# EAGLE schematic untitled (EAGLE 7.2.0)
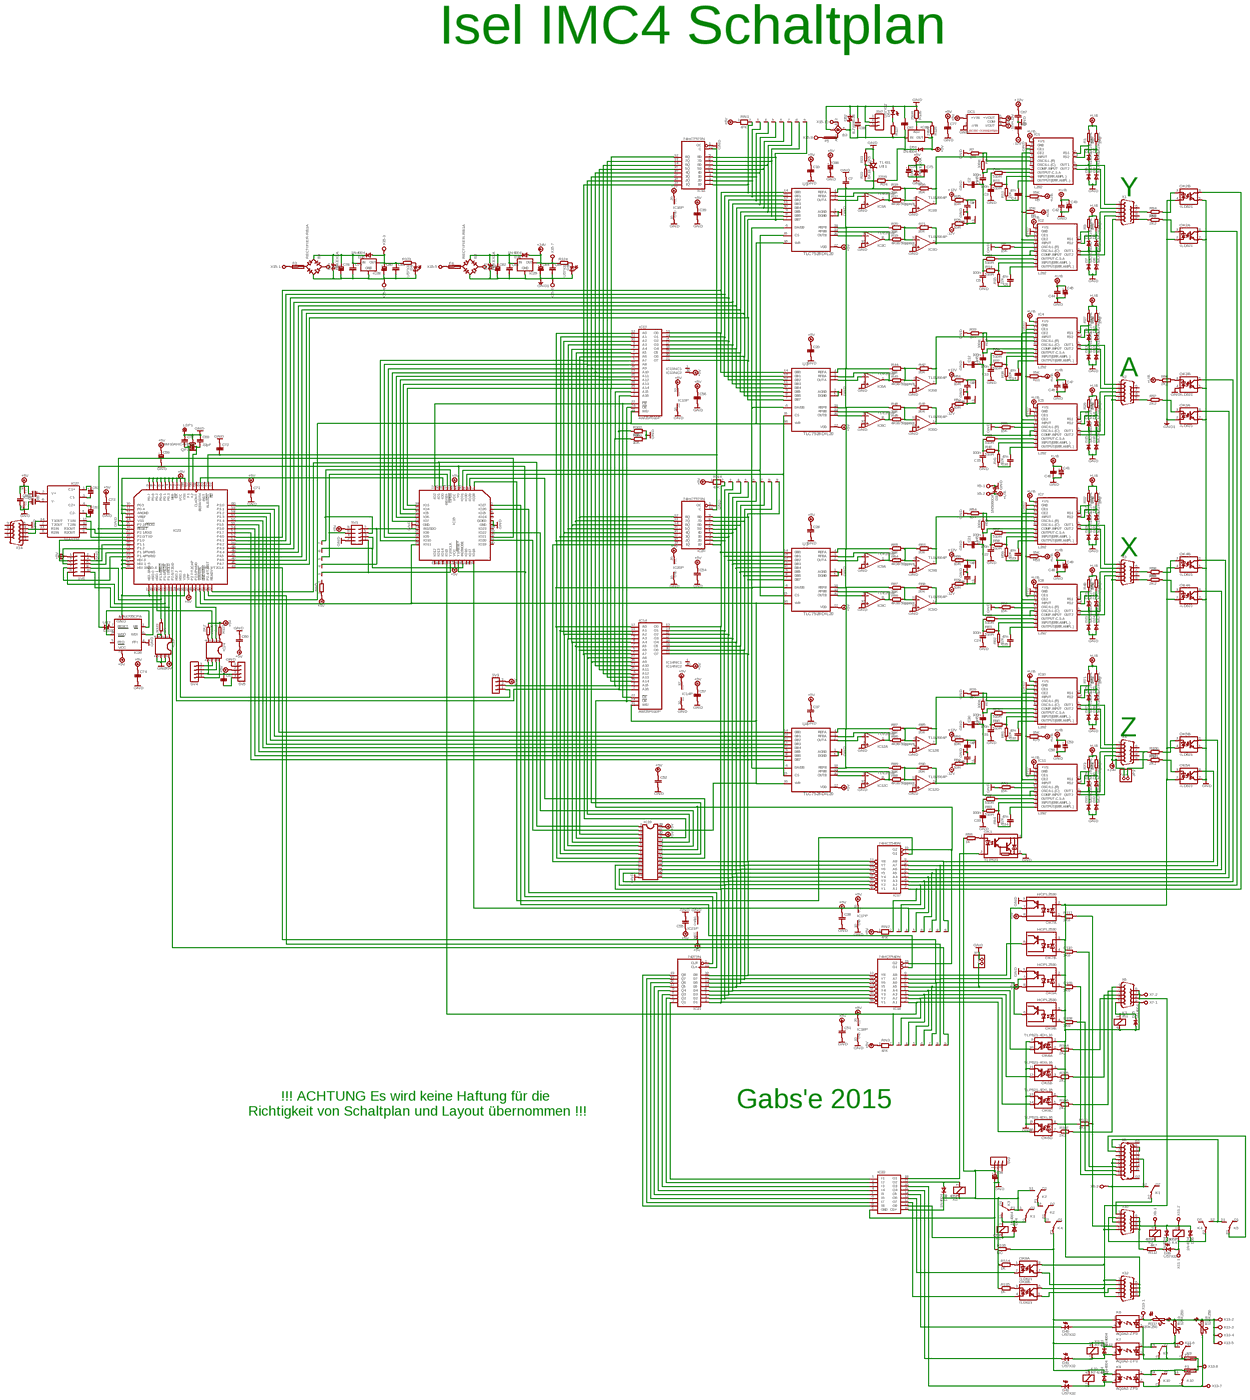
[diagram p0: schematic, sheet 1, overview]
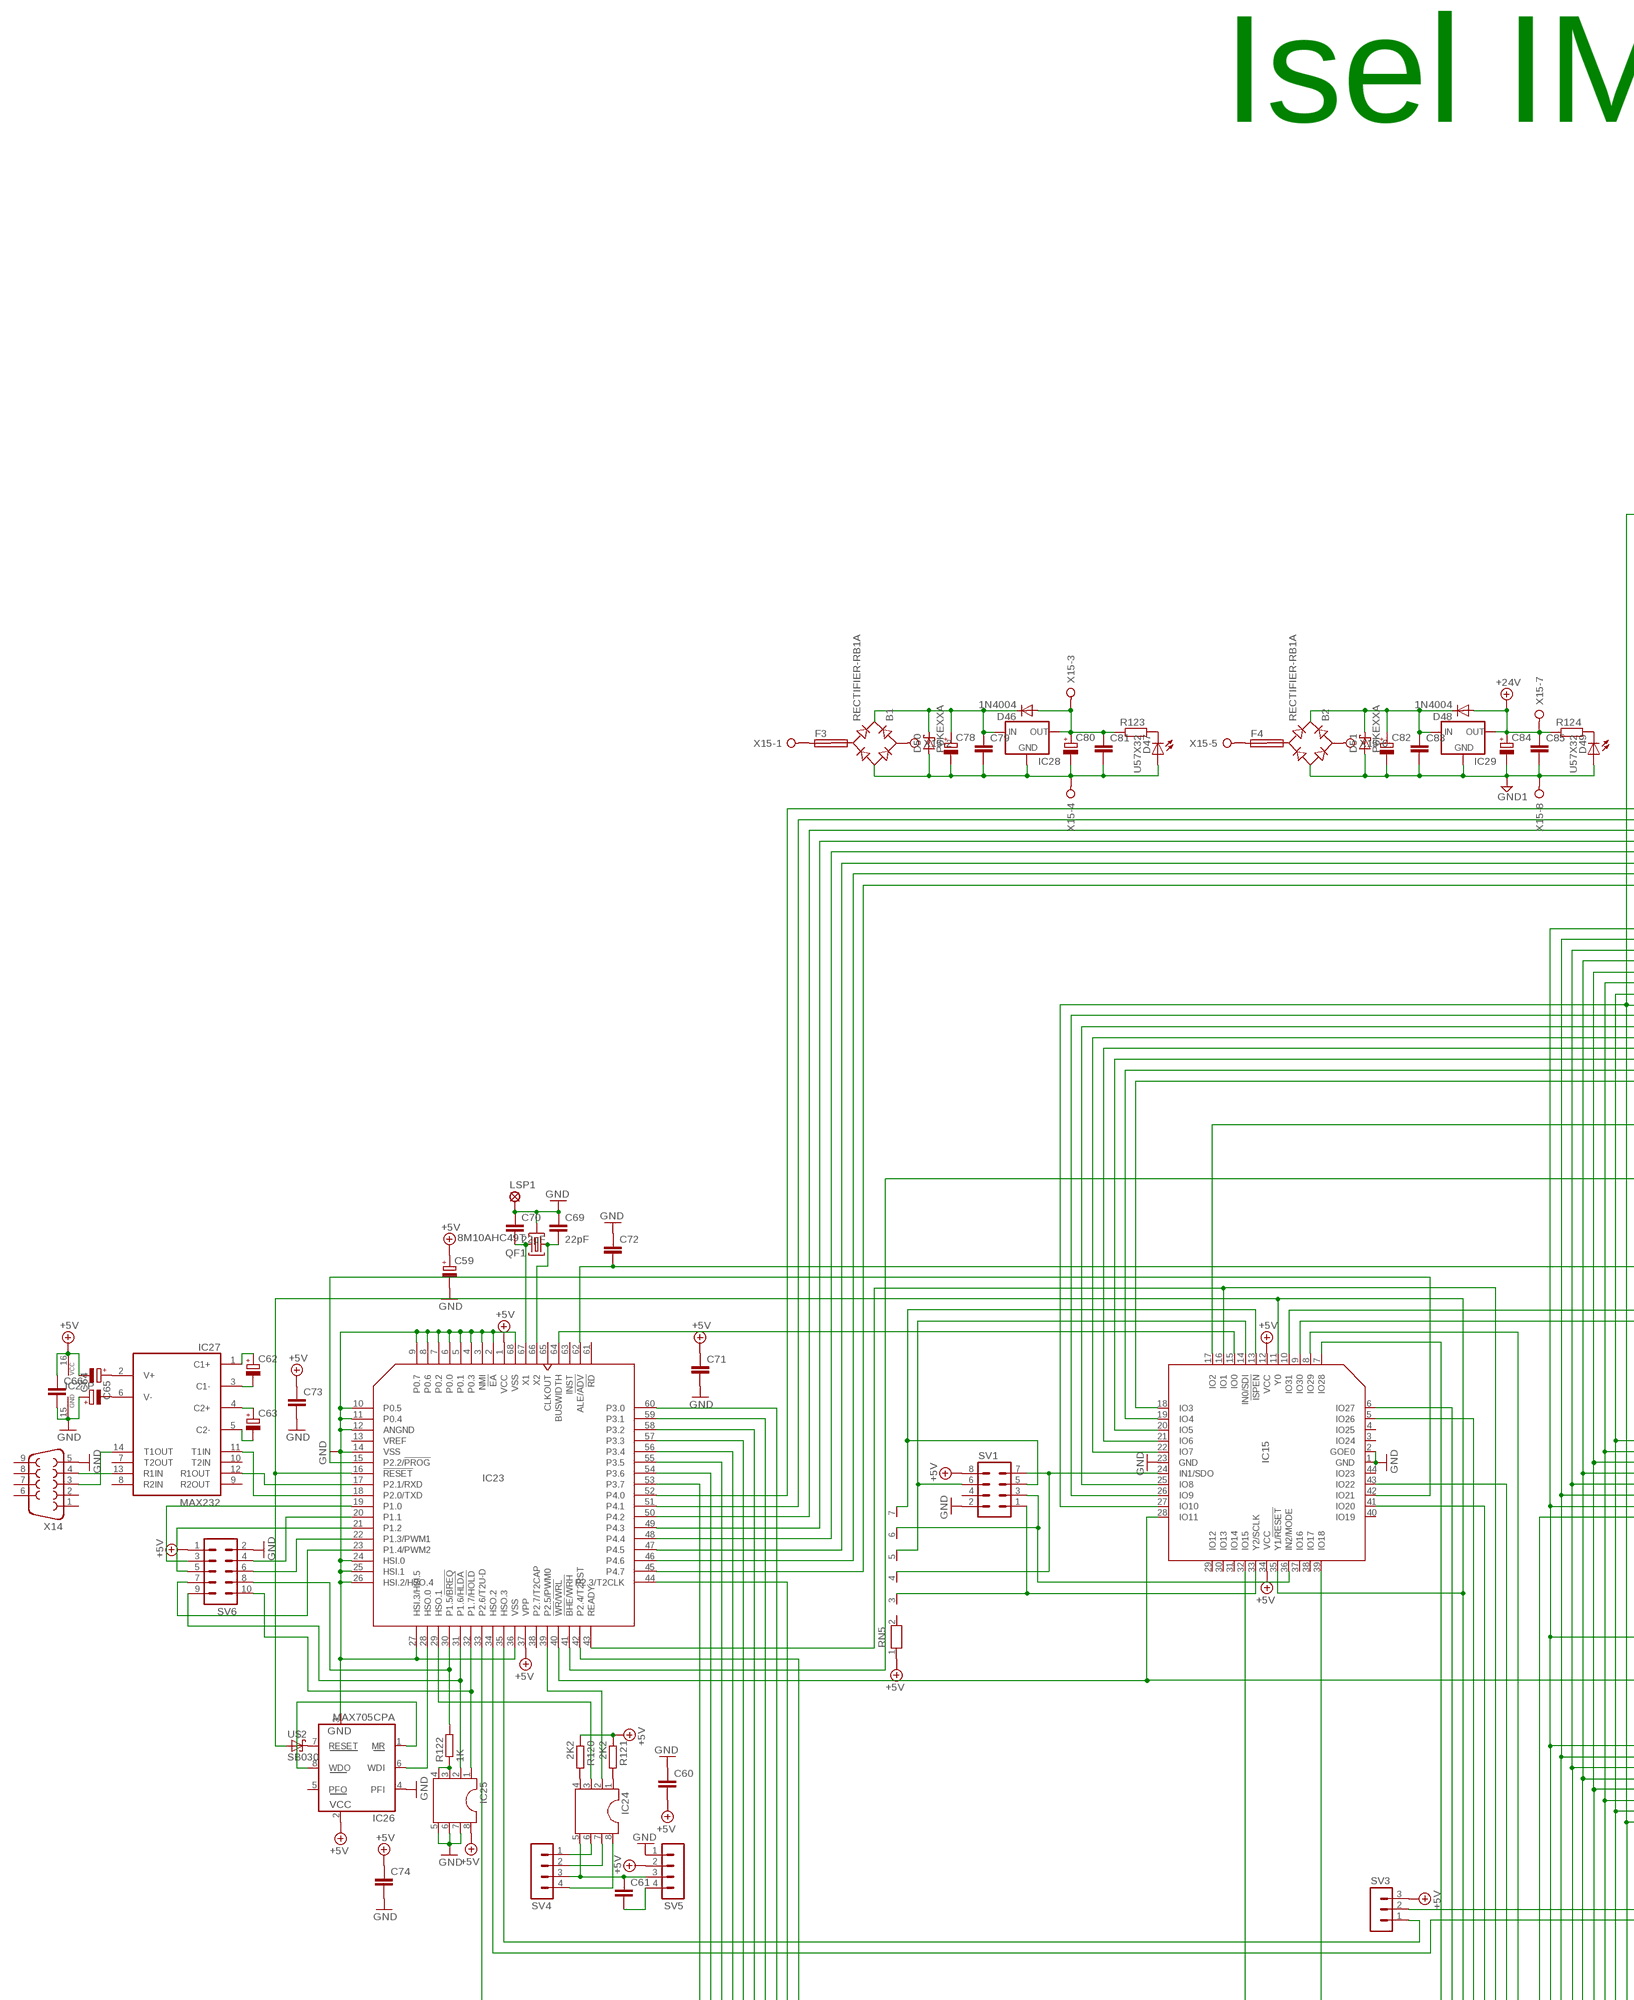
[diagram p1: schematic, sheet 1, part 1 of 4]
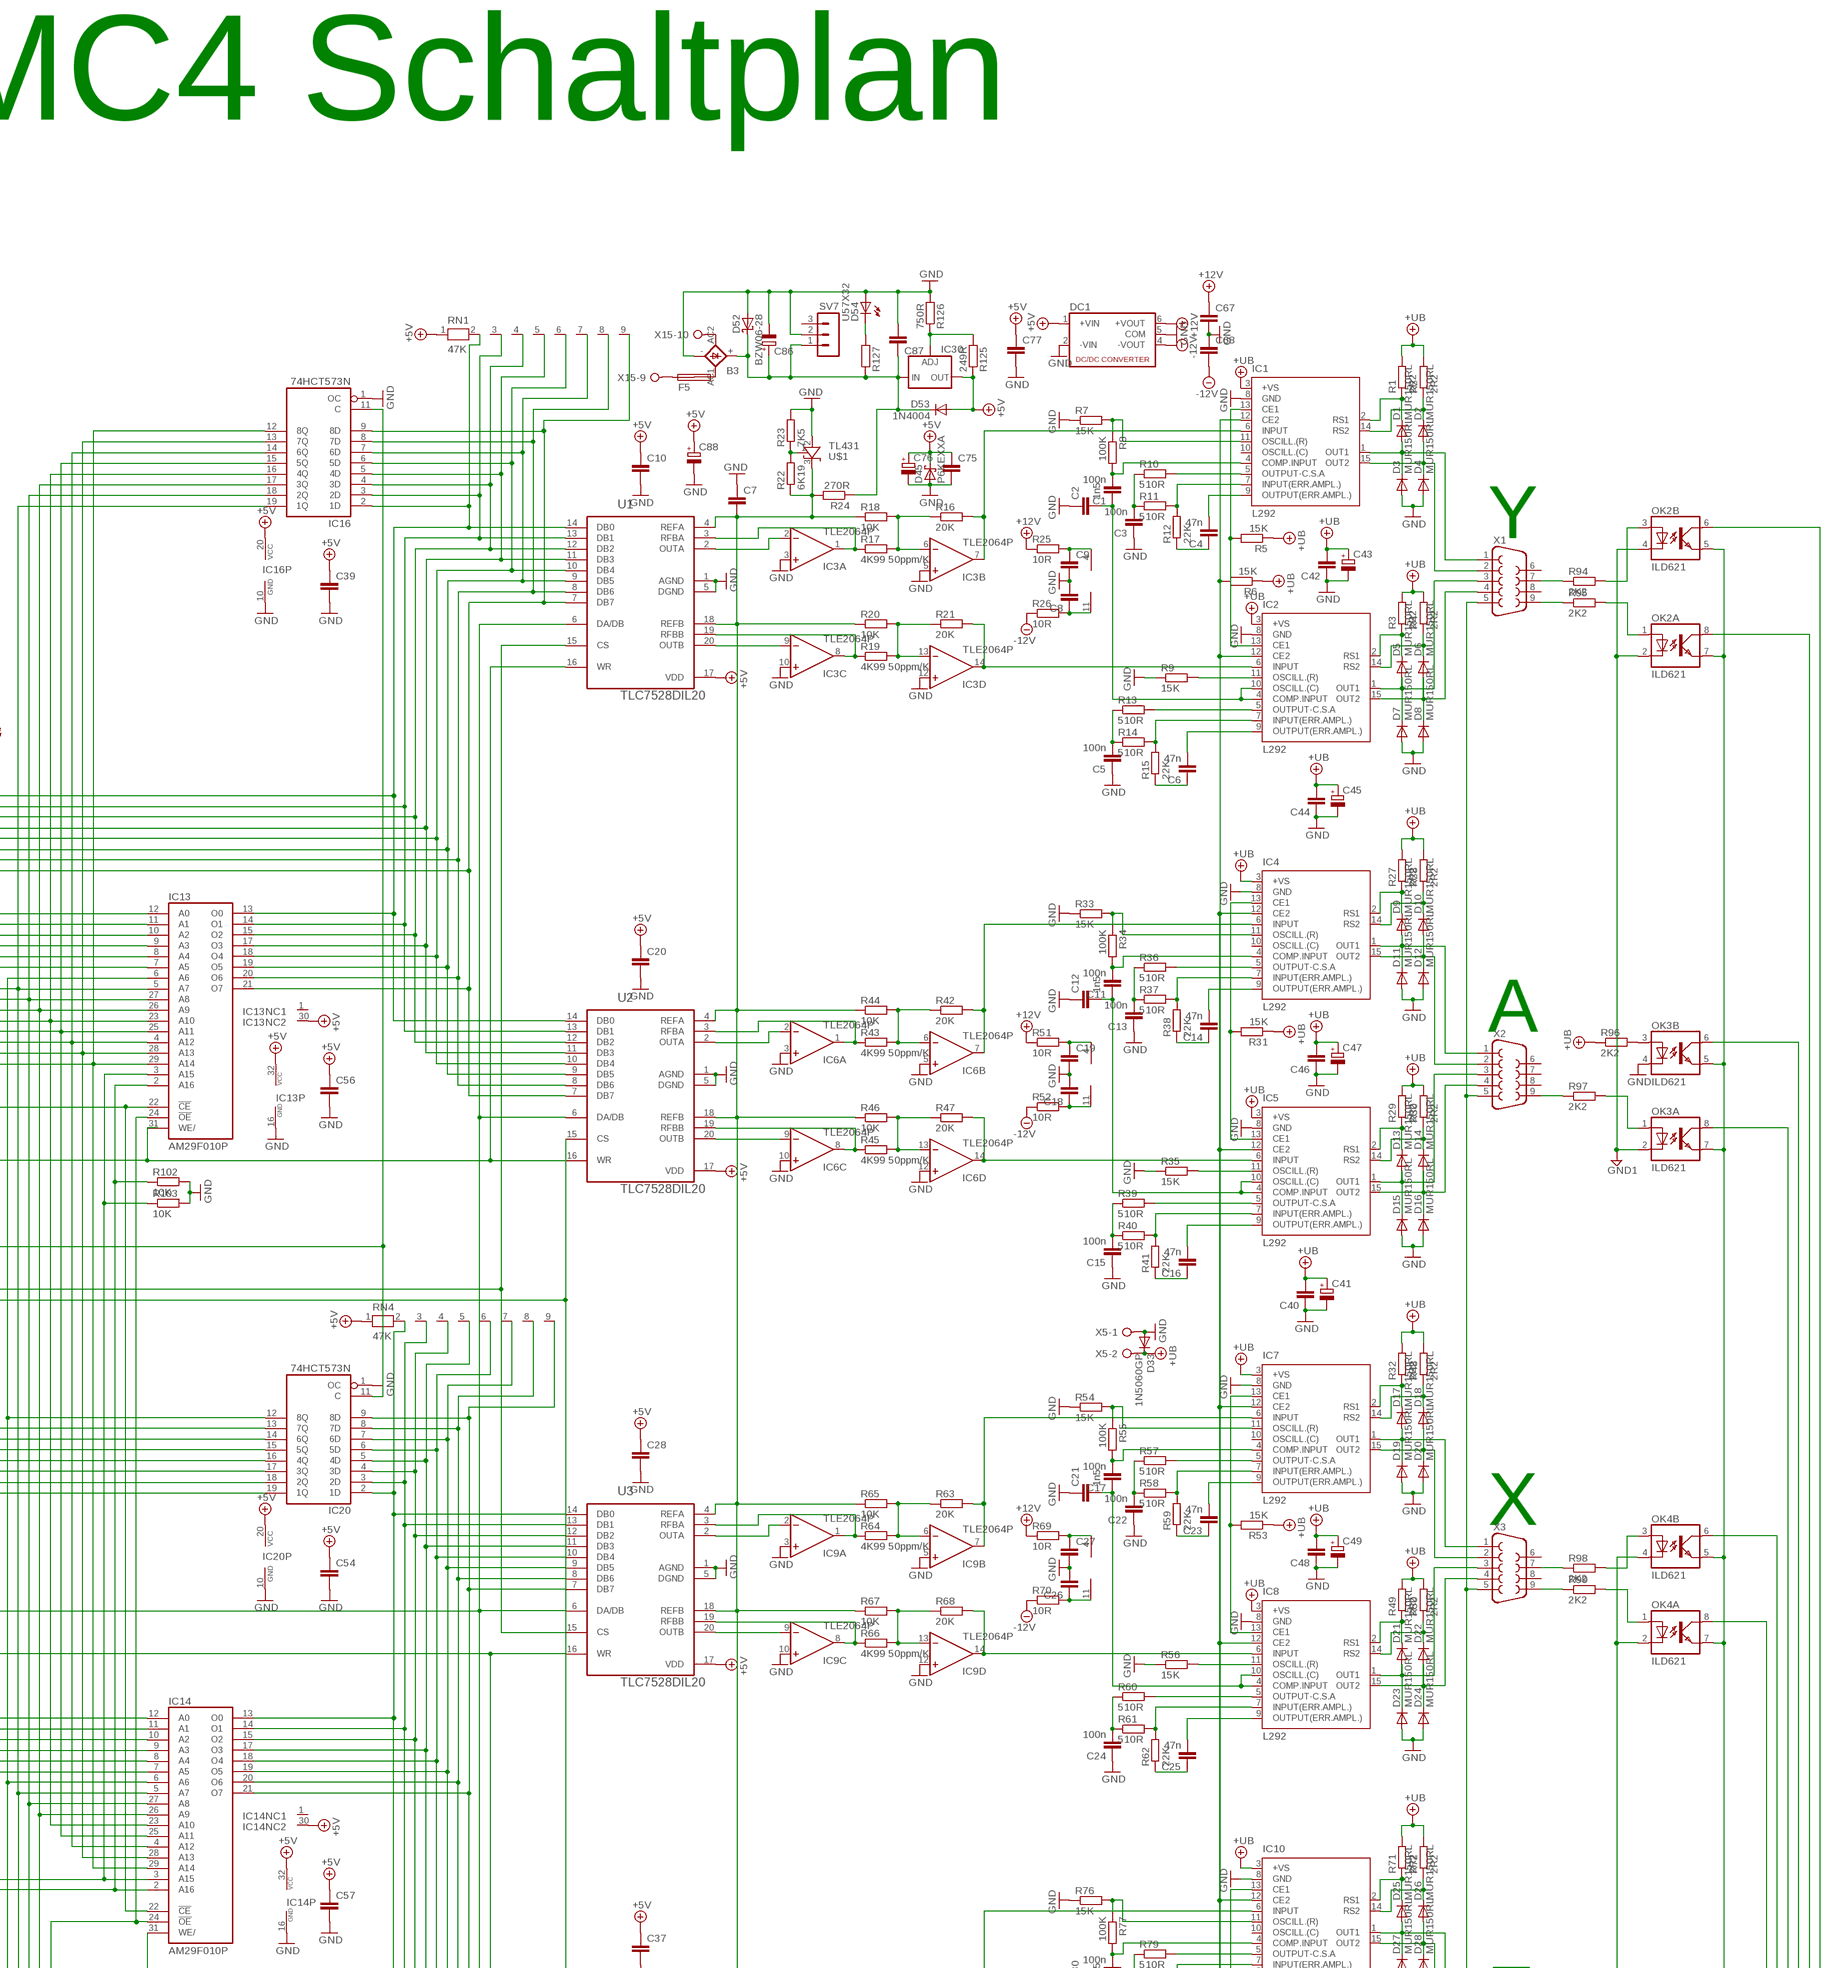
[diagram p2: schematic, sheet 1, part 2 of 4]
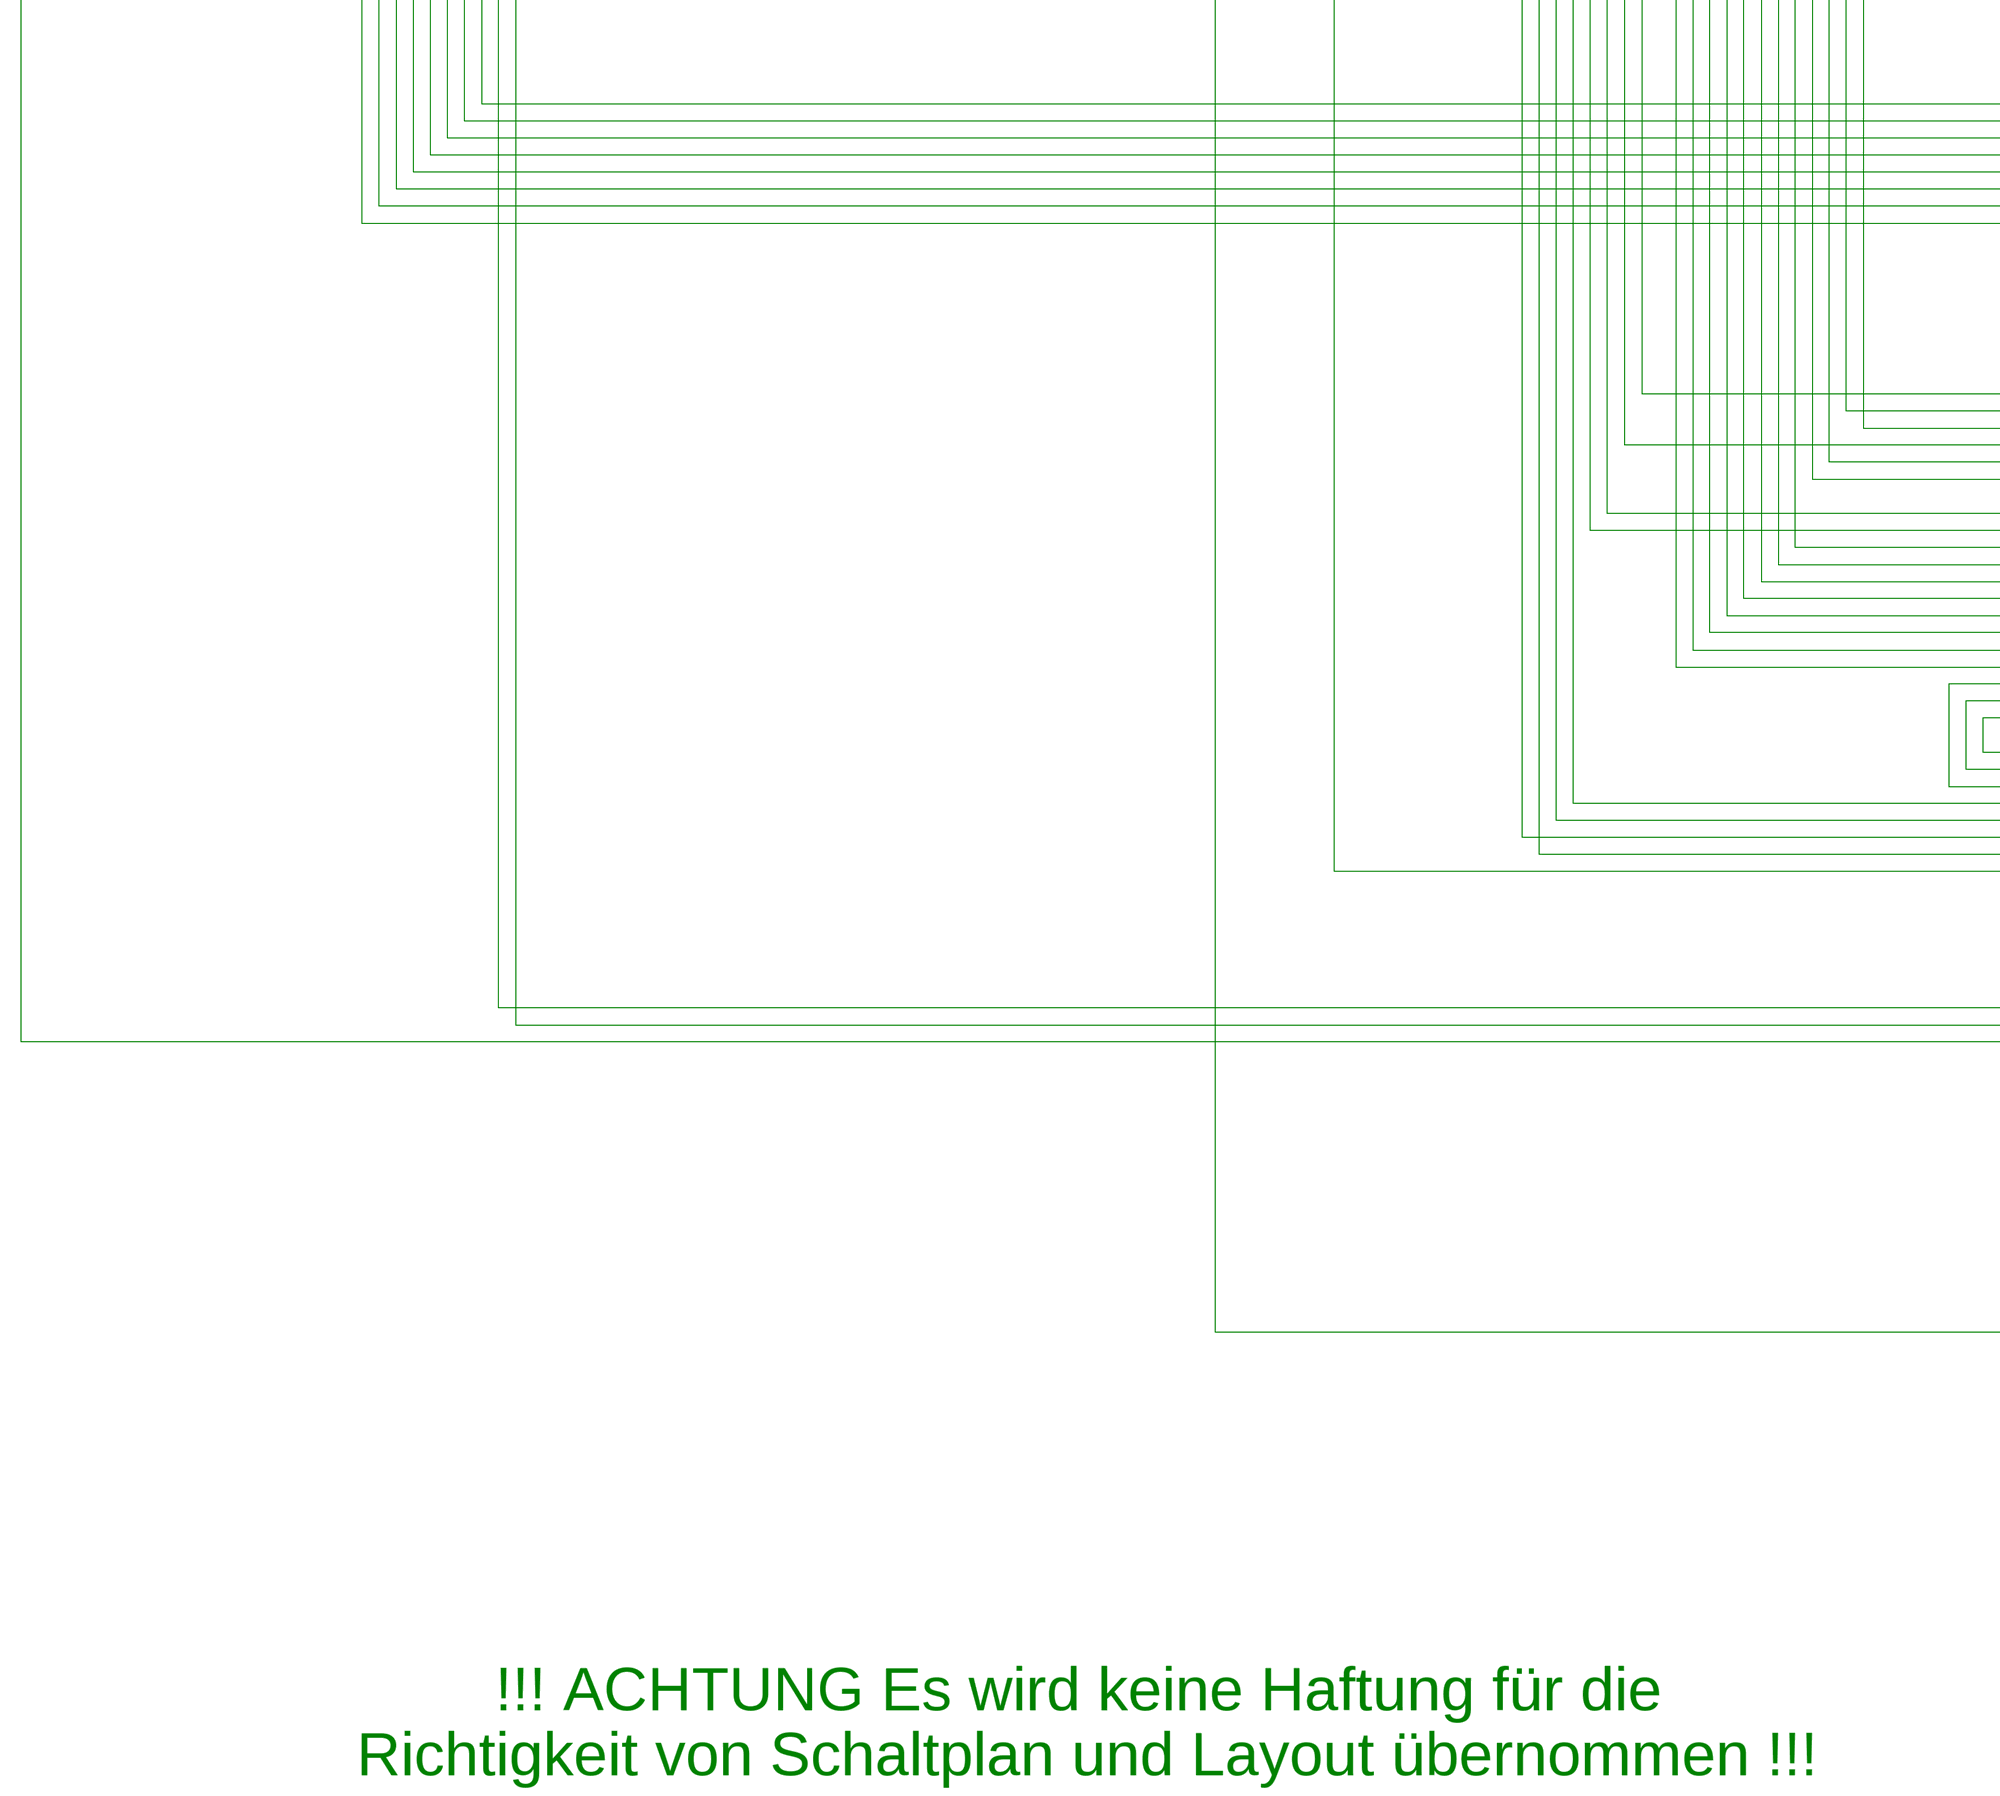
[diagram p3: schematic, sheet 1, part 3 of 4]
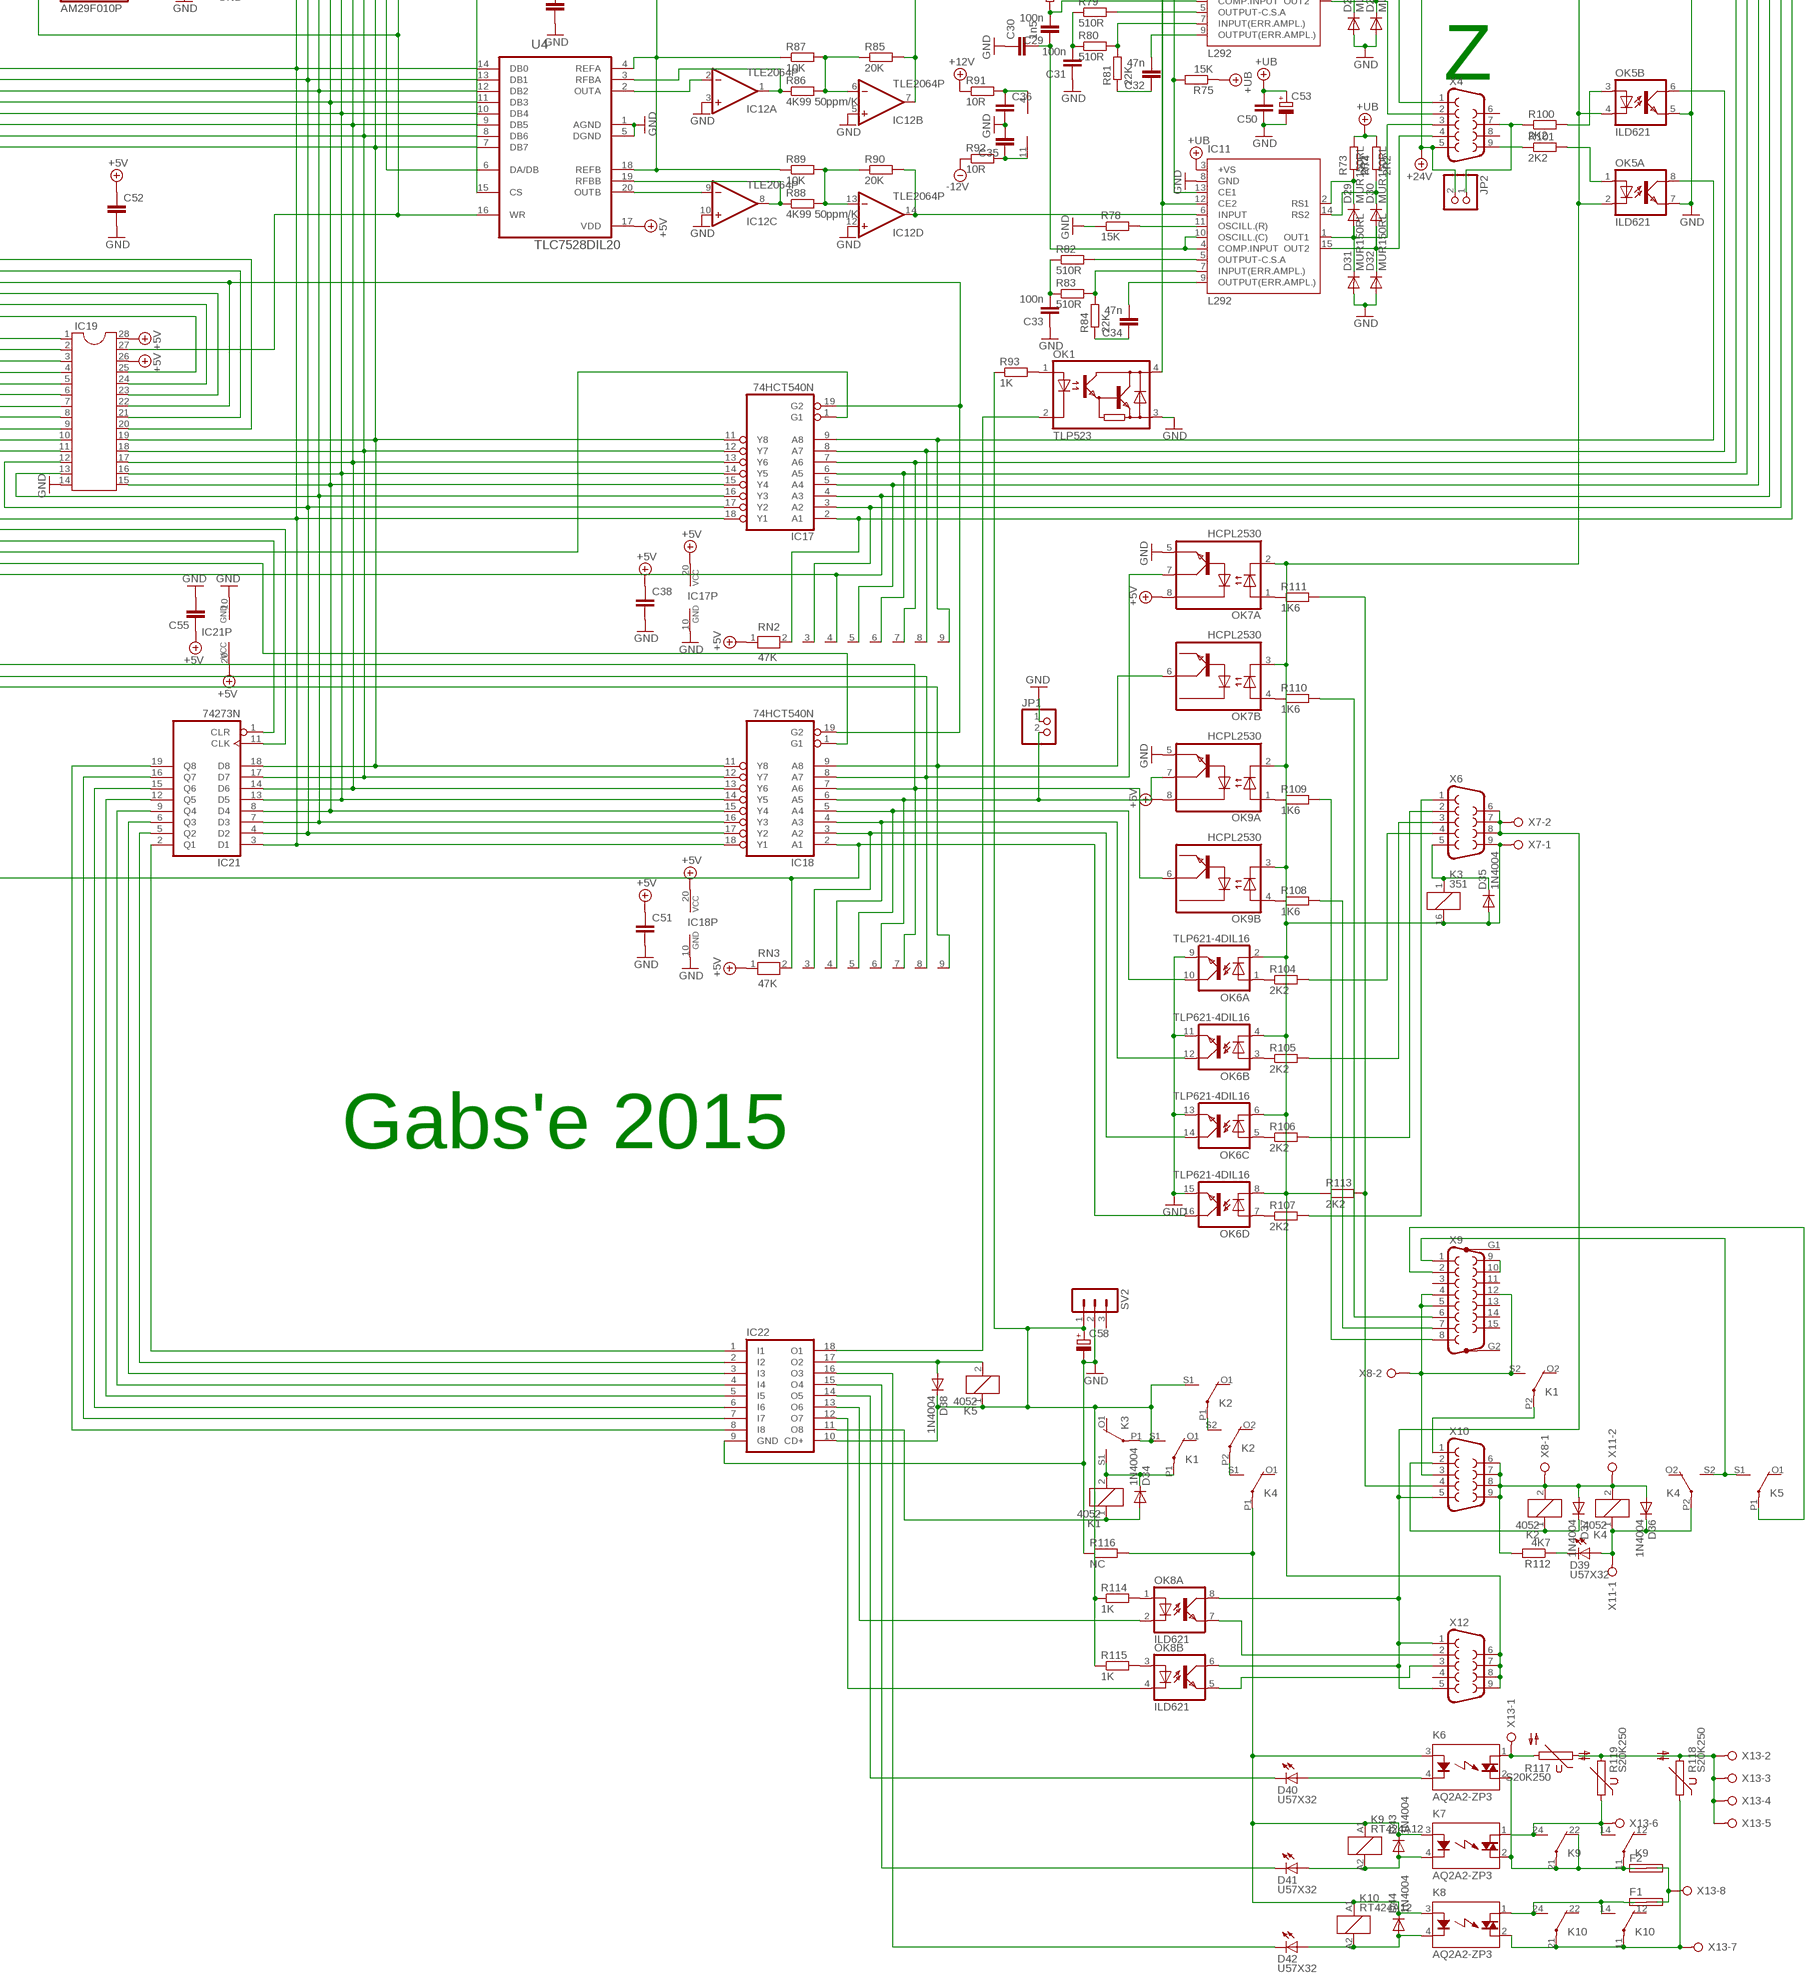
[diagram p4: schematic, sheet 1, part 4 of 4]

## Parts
B1  RECTIFIER-RB1A  [RB1A]
B2  RECTIFIER-RB1A  [RB1A]
B3  2KBB-R  [2KBB-R]
C1  100n  C-EU050-025X075  [C050-025X075]
C2  1n5  C-EU050-025X075  [C050-025X075]
C3  100n  C-EU050-025X075  [C050-025X075]
C4  47n  C-EU050-025X075  [C050-025X075]
C5  100n  C-EU050-025X075  [C050-025X075]
C6  47n  C-EU050-025X075  [C050-025X075]
C7  C-EU025-024X044  [C025-024X044]
C8  C-EU025-024X044  [C025-024X044]
C9  C-EU025-024X044  [C025-024X044]
C10  C-EU025-024X044  [C025-024X044]
C11  100n  C-EU050-025X075  [C050-025X075]
C12  1n5  C-EU050-025X075  [C050-025X075]
C13  100n  C-EU050-025X075  [C050-025X075]
C14  47n  C-EU050-025X075  [C050-025X075]
C15  100n  C-EU050-025X075  [C050-025X075]
C16  47n  C-EU050-025X075  [C050-025X075]
C17  100n  C-EU050-025X075  [C050-025X075]
C18  C-EU025-024X044  [C025-024X044]
C19  C-EU025-024X044  [C025-024X044]
C20  C-EU025-024X044  [C025-024X044]
C21  1n5  C-EU050-025X075  [C050-025X075]
C22  100n  C-EU050-025X075  [C050-025X075]
C23  47n  C-EU050-025X075  [C050-025X075]
C24  100n  C-EU050-025X075  [C050-025X075]
C25  47n  C-EU050-025X075  [C050-025X075]
C26  C-EU025-024X044  [C025-024X044]
C27  C-EU025-024X044  [C025-024X044]
C28  C-EU025-024X044  [C025-024X044]
C29  100n  C-EU050-025X075  [C050-025X075]
C30  1n5  C-EU050-025X075  [C050-025X075]
C31  100n  C-EU050-025X075  [C050-025X075]
C32  47n  C-EU050-025X075  [C050-025X075]
C33  100n  C-EU050-025X075  [C050-025X075]
C34  47n  C-EU050-025X075  [C050-025X075]
C35  C-EU025-024X044  [C025-024X044]
C36  C-EU025-024X044  [C025-024X044]
C37  C-EU025-024X044  [C025-024X044]
C38  C-EU025-024X044  [C025-024X044]
C39  C-EU025-024X044  [C025-024X044]
C40  C-EU025-024X044  [C025-024X044]
C41  CPOL-EUE2.5-6  [E2,5-6]
C42  C-EU050-025X075  [C050-025X075]
C43  CPOL-EUE2,5-6E  [E2,5-6E]
C44  C-EU050-025X075  [C050-025X075]
C45  CPOL-EUE2.5-6  [E2,5-6]
C46  C-EU050-025X075  [C050-025X075]
C47  CPOL-EUE2.5-6  [E2,5-6]
C48  C-EU050-025X075  [C050-025X075]
C49  CPOL-EUE2.5-6  [E2,5-6]
C50  C-EU050-025X075  [C050-025X075]
C51  C-EU025-024X044  [C025-024X044]
C52  C-EU025-024X044  [C025-024X044]
C53  CPOL-EUE2.5-6  [E2,5-6]
C54  C-EU025-024X044  [C025-024X044]
C55  C-EU025-024X044  [C025-024X044]
C56  C-EU025-024X044  [C025-024X044]
C57  C-EU025-024X044  [C025-024X044]
C58  CPOL-EUE1.8-4  [E1,8-4]
C59  CPOL-EUE2.5-6  [E2,5-6]
C60  C-EU025-024X044  [C025-024X044]
C61  C-EU025-024X044  [C025-024X044]
C62  CPOL-EUE2.5-6  [E2,5-6]
C63  CPOL-EUE2.5-6  [E2,5-6]
C64  CPOL-EUE2,5-6E  [E2,5-6E]
C65  CPOL-EUE2.5-6  [E2,5-6]
C66  C-EU025-024X044  [C025-024X044]
C67  C-EU025-024X044  [C025-024X044]
C68  C-EU025-024X044  [C025-024X044]
C69  22pF  C-EU025-024X044  [C025-024X044]
C70  22pF  C-EU025-024X044  [C025-024X044]
C71  C-EU025-024X044  [C025-024X044]
C72  C-EU025-024X044  [C025-024X044]
C73  C-EU025-024X044  [C025-024X044]
C74  C-EU025-024X044  [C025-024X044]
C75  C-EU025-024X044  [C025-024X044]
C76  CPOL-EUE2.5-6  [E2,5-6]
C77  C-EU025-024X044  [C025-024X044]
C78  CPOL-EUE7.5-16  [E7,5-16]
C79  C-EU025-024X044  [C025-024X044]
C80  CPOL-EUE2-5  [E2-5]
C81  C-EU025-024X044  [C025-024X044]
C82  CPOL-EUE7.5-16  [E7,5-16]
C83  C-EU025-024X044  [C025-024X044]
C84  CPOL-EUE2-5  [E2-5]
C85  C-EU025-024X044  [C025-024X044]
C86  CPOL-EUE7.5-16  [E7,5-16]
C87  C-EU025-024X044  [C025-024X044]
C88  CPOL-EUE2.5-6  [E2,5-6]
D1  MUR150RL  [DO41-10]
D2  MUR150RL  [DO41-10]
D3  MUR150RL  [DO41-10]
D4  MUR150RL  [DO41-10]
D5  MUR150RL  [DO41-10]
D6  MUR150RL  [DO41-10]
D7  MUR150RL  [DO41-10]
D8  MUR150RL  [DO41-10]
D9  MUR150RL  [DO41-10]
D10  MUR150RL  [DO41-10]
D11  MUR150RL  [DO41-10]
D12  MUR150RL  [DO41-10]
D13  MUR150RL  [DO41-10]
D14  MUR150RL  [DO41-10]
D15  MUR150RL  [DO41-10]
D16  MUR150RL  [DO41-10]
D17  MUR150RL  [DO41-10]
D18  MUR150RL  [DO41-10]
D19  MUR150RL  [DO41-10]
D20  MUR150RL  [DO41-10]
D21  MUR150RL  [DO41-10]
D22  MUR150RL  [DO41-10]
D23  MUR150RL  [DO41-10]
D24  MUR150RL  [DO41-10]
D25  MUR150RL  [DO41-10]
D26  MUR150RL  [DO41-10]
D27  MUR150RL  [DO41-10]
D28  MUR150RL  [DO41-10]
D29  MUR150RL  [DO41-10]
D30  MUR150RL  [DO41-10]
D31  MUR150RL  [DO41-10]
D32  MUR150RL  [DO41-10]
D33  1N5060GP  [DO15-12]
D34  1N4004  [DO41-10]
D35  1N4004  [DO41-10]
D36  1N4004  [DO41-10]
D37  1N4004  [DO41-10]
D38  1N4004  [DO41-10]
D39  U57X32  [U57X32]
D40  U57X32  [U57X32]
D41  U57X32  [U57X32]
D42  U57X32  [U57X32]
D43  1N4004  [DO41-10]
D44  1N4004  [DO41-10]
D45  P6KEXXA  [C1702-15]
D46  1N4004  [DO41-10]
D47  U57X32  [U57X32]
D48  1N4004  [DO41-10]
D49  U57X32  [U57X32]
D50  P6KEXXA  [C1702-15]
D51  P6KEXXA  [C1702-15]
D52  BZW06-28  [P1-12E]
D53  1N4004  [DO41-10]
D54  U57X32  [U57X32]
DC1  NMA  [NMA]
F1  SHK20L  [SHK20L]
F2  SHK20L  [SHK20L]
F3  SHK20L  [SHK20L]
F4  SHK20L  [SHK20L]
F5  SHK20L  [SHK20L]
IC1  L292  [MULTIWATT-15]
IC2  L292  [MULTIWATT-15]
IC3  TLE2064P  [DIL14]
IC4  L292  [MULTIWATT-15]
IC5  L292  [MULTIWATT-15]
IC6  TLE2064P  [DIL14]
IC7  L292  [MULTIWATT-15]
IC8  L292  [MULTIWATT-15]
IC9  TLE2064P  [DIL14]
IC10  L292  [MULTIWATT-15]
IC11  L292  [MULTIWATT-15]
IC12  TLE2064P  [DIL14]
IC13  AM29F010P  [DIL32-3]
IC14  AM29F010P  [DIL32-3]
IC15  LSI2032PLCC  [S44]
IC16  74HCT573N  [DIL20]
IC17  74HCT540N  [DIL20]
IC18  74HCT540N  [DIL20]
IC19  DIL28  [DIL28-6]
IC20  74HCT573N  [DIL20]
IC21  74273N  [DIL20]
IC22  ULN2803A  [DIL18]
IC23  N80C196KC  [S68]
IC24  DIL8  [DIL08]
IC25  DIL8  [DIL08]
IC26  MAX705CPA  [DIL08]
IC27  MAX232  [DIL16]
IC28  78XXS  [78XXS]
IC29  78XXS  [78XXS]
IC30  LM317TS  [317TS]
JP1  PINHD-1X2  [1X02]
JP2  PINHD-1X2  [1X02]
K1  4052  [F4052]
K2  4052  [F4052]
K3  351  [351]
K4  4052  [F4052]
K5  4052  [F4052]
K6  AQ2A2-ZP3  [AQ1]
K7  AQ2A2-ZP3  [AQ1]
K8  AQ2A2-ZP3  [AQ1]
K9  RT424A12  [RT2C/O]
K10  RT424A12  [RT2C/O]
LSP1  LSP10  [LSP10]
OK1  TLP523  [DIL04]
OK2  ILD621  [DIL08]
OK3  ILD621  [DIL08]
OK4  ILD621  [DIL08]
OK5  ILD621  [DIL08]
OK6  TLP621-4DIL16  [DIL16]
OK7  HCPL2530  [DIL08]
OK8  ILD621  [DIL08]
OK9  HCPL2530  [DIL08]
QF1  8M10AHC49T  [HC49U]
R1  2R2  R-EU_0411/15  [0411/15]
R2  2R2  R-EU_0411/15  [0411/15]
R3  2R2  R-EU_0411/15  [0411/15]
R4  2R2  R-EU_0411/15  [0411/15]
R5  15K  R-EU_V526-0  [V526-0]
R6  15K  R-EU_V526-0  [V526-0]
R7  15K  R-EU_V526-0  [V526-0]
R8  100K  R-EU_V526-0  [V526-0]
R9  15K  R-EU_V526-0  [V526-0]
R10  510R  R-EU_V526-0  [V526-0]
R11  510R  R-EU_V526-0  [V526-0]
R12  22K  R-EU_V526-0  [V526-0]
R13  510R  R-EU_V526-0  [V526-0]
R14  510R  R-EU_V526-0  [V526-0]
R15  22K  R-EU_V526-0  [V526-0]
R16  20K  R-EU_0207/10  [0207/10]
R17  4K99 50ppm/K  R-EU_0207/10  [0207/10]
R18  10K  R-EU_0207/10  [0207/10]
R19  4K99 50ppm/K  R-EU_0207/10  [0207/10]
R20  10K  R-EU_0207/10  [0207/10]
R21  20K  R-EU_0207/10  [0207/10]
R22  6K19  R-EU_0207/10  [0207/10]
R23  7K5  R-EU_0207/10  [0207/10]
R24  270R  R-EU_0207/10  [0207/10]
R25  10R  R-EU_V526-0  [V526-0]
R26  10R  R-EU_V526-0  [V526-0]
R27  2R2  R-EU_0411/15  [0411/15]
R28  2R2  R-EU_0411/15  [0411/15]
R29  2R2  R-EU_0411/15  [0411/15]
R30  2R2  R-EU_0411/15  [0411/15]
R31  15K  R-EU_V526-0  [V526-0]
R32  2R2  R-EU_0411/15  [0411/15]
R33  15K  R-EU_V526-0  [V526-0]
R34  100K  R-EU_V526-0  [V526-0]
R35  15K  R-EU_V526-0  [V526-0]
R36  510R  R-EU_V526-0  [V526-0]
R37  510R  R-EU_V526-0  [V526-0]
R38  22K  R-EU_V526-0  [V526-0]
R39  510R  R-EU_V526-0  [V526-0]
R40  510R  R-EU_V526-0  [V526-0]
R41  22K  R-EU_V526-0  [V526-0]
R42  20K  R-EU_0207/10  [0207/10]
R43  4K99 50ppm/K  R-EU_0207/10  [0207/10]
R44  10K  R-EU_0207/10  [0207/10]
R45  4K99 50ppm/K  R-EU_0207/10  [0207/10]
R46  10K  R-EU_0207/10  [0207/10]
R47  20K  R-EU_0207/10  [0207/10]
R48  2R2  R-EU_0411/15  [0411/15]
R49  2R2  R-EU_0411/15  [0411/15]
R50  2R2  R-EU_0411/15  [0411/15]
R51  10R  R-EU_V526-0  [V526-0]
R52  10R  R-EU_V526-0  [V526-0]
R53  15K  R-EU_V526-0  [V526-0]
R54  15K  R-EU_V526-0  [V526-0]
R55  100K  R-EU_V526-0  [V526-0]
R56  15K  R-EU_V526-0  [V526-0]
R57  510R  R-EU_V526-0  [V526-0]
R58  510R  R-EU_V526-0  [V526-0]
R59  22K  R-EU_V526-0  [V526-0]
R60  510R  R-EU_V526-0  [V526-0]
R61  510R  R-EU_V526-0  [V526-0]
R62  22K  R-EU_V526-0  [V526-0]
R63  20K  R-EU_0207/10  [0207/10]
R64  4K99 50ppm/K  R-EU_0207/10  [0207/10]
R65  10K  R-EU_0207/10  [0207/10]
R66  4K99 50ppm/K  R-EU_0207/10  [0207/10]
R67  10K  R-EU_0207/10  [0207/10]
R68  20K  R-EU_0207/10  [0207/10]
R69  10R  R-EU_V526-0  [V526-0]
R70  10R  R-EU_V526-0  [V526-0]
R71  2R2  R-EU_0411/15  [0411/15]
R72  2R2  R-EU_0411/15  [0411/15]
R73  2R2  R-EU_0411/15  [0411/15]
R74  2R2  R-EU_0411/15  [0411/15]
R75  15K  R-EU_V526-0  [V526-0]
R76  15K  R-EU_V526-0  [V526-0]
R77  100K  R-EU_V526-0  [V526-0]
R78  15K  R-EU_V526-0  [V526-0]
R79  510R  R-EU_V526-0  [V526-0]
R80  510R  R-EU_V526-0  [V526-0]
R81  22K  R-EU_V526-0  [V526-0]
R82  510R  R-EU_V526-0  [V526-0]
R83  510R  R-EU_V526-0  [V526-0]
R84  22K  R-EU_V526-0  [V526-0]
R85  20K  R-EU_0207/10  [0207/10]
R86  4K99 50ppm/K  R-EU_0207/10  [0207/10]
R87  10K  R-EU_0207/10  [0207/10]
R88  4K99 50ppm/K  R-EU_0207/10  [0207/10]
R89  10K  R-EU_0207/10  [0207/10]
R90  20K  R-EU_0207/10  [0207/10]
R91  10R  R-EU_V526-0  [V526-0]
R92  10R  R-EU_V526-0  [V526-0]
R93  1K  R-EU_V526-0  [V526-0]
R94  2K2  R-EU_V526-0  [V526-0]
R95  2K2  R-EU_V526-0  [V526-0]
R96  2K2  R-EU_V526-0  [V526-0]
R97  2K2  R-EU_V526-0  [V526-0]
R98  2K2  R-EU_V526-0  [V526-0]
R99  2K2  R-EU_V526-0  [V526-0]
R100  2K2  R-EU_V526-0  [V526-0]
R101  2K2  R-EU_V526-0  [V526-0]
R102  10K  R-EU_0207/10  [0207/10]
R103  10K  R-EU_0207/10  [0207/10]
R104  2K2  R-EU_V526-0  [V526-0]
R105  2K2  R-EU_V526-0  [V526-0]
R106  2K2  R-EU_V526-0  [V526-0]
R107  2K2  R-EU_V526-0  [V526-0]
R108  1K6  R-EU_V526-0  [V526-0]
R109  1K6  R-EU_V526-0  [V526-0]
R110  1K6  R-EU_V526-0  [V526-0]
R111  1K6  R-EU_V526-0  [V526-0]
R112  4K7  R-EU_0207/10  [0207/10]
R113  2K2  R-EU_V526-0  [V526-0]
R114  1K  R-EU_V526-0  [V526-0]
R115  1K  R-EU_V526-0  [V526-0]
R116  NC  R-EU_V526-0  [V526-0]
R117  S20K250  [S20K250]
R118  S20K250  [S20K250]
R119  S20K250  [S20K250]
R120  2K2  R-EU_V526-0  [V526-0]
R121  2K2  R-EU_V526-0  [V526-0]
R122  1K  R-EU_V526-0  [V526-0]
R123  R-EU_0207/10  [0207/10]
R124  R-EU_0207/10  [0207/10]
R125  249R  R-EU_0207/10  [0207/10]
R126  750R  R-EU_0207/10  [0207/10]
R127  R-EU_0207/10  [0207/10]
RN1  47K  RN08  [RN-9]
RN2  47K  RN08  [RN-9]
RN3  47K  RN08  [RN-9]
RN4  47K  RN08  [RN-9]
RN5  RN06  [RN-7]
SV1  MA04-2  [MA04-2]
SV2  MA03-1  [MA03-1]
SV3  MA03-1  [MA03-1]
SV4  MA04-1  [MA04-1]
SV5  MA04-1  [MA04-1]
SV6  MA05-2  [MA05-2]
SV7  MA03-1  [MA03-1]
U1  TLC7528DIL20  [DIL20]
U2  TLC7528DIL20  [DIL20]
U3  TLC7528DIL20  [DIL20]
U4  TLC7528DIL20  [DIL20]
U$1  TL431  [TO-92]
U$2  SB030  [DO41-10]
X1  F09HP  [F09HP]
X2  F09HP  [F09HP]
X3  F09HP  [F09HP]
X4  F09HP  [F09HP]
X5  W237-02P  [W237-132]
X6  F09VP  [F09VP]
X7  W237-02P  [W237-132]
X8  W237-02P  [W237-132]
X9  F15VP  [F15VP]
X10  F09VP  [F09VP]
X11  W237-02P  [W237-132]
X12  F09VP  [F09VP]
X13  W237-08P  [W237-8P]
X14  F09VP  [F09VP]
X15  W237-10P  [W237-10P]

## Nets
+5V: C10.1 C20.1 C28.1 C37.1 C38.1 C39.1 C51.1 C52.1 C54.1 C55.1 C56.1 C57.1 C59.+ C60.2 C65.- C66.1 C71.1 C73.1 C74.1 C75.1 C76.+ C77.1 C88.+ D45.C D53.A DC1.1(+VIN) IC13.30(NC) IC13.32(VCC) IC14.30(NC) IC14.32(VCC) IC15.12(VCC) IC15.34(VCC) IC16.20(VCC) IC17.20(VCC) IC18.20(VCC) IC19.26 IC19.28 IC20.20(VCC) IC21.20(VCC) IC23.1(VCC) IC23.37(VPP) IC25.8 IC26.2(VCC) IC27.16(VCC) IC30.2(OUT) OK7.8(A:VCC) OK9.8(A:VCC) R120.1 R121.1 R125.1 RN1.1 RN2.1 RN3.1 RN4.1 RN5.1 SV1.8 SV3.3 SV5.2 SV6.1 U1.17(VDD) U2.17(VDD) U3.17(VDD) U4.17(VDD)
+12V: C67.1 DC1.6(+VOUT) R25.1 R51.1 R69.1 R91.1
+24V: C84.+ C85.1 D48.A IC29.OUT JP2.2 R124.1 X1.5 X2.5 X3.5 X4.5 X15.7
+UB: C40.2 C41.+ C42.2 C43.+ C44.2 C45.+ C46.2 C47.+ C48.2 C49.+ C50.2 C53.+ D33.C IC1.3(+VS) IC2.3(+VS) IC4.3(+VS) IC5.3(+VS) IC7.3(+VS) IC8.3(+VS) IC10.3(+VS) IC11.3(+VS) R1.2 R2.2 R3.2 R4.2 R5.1 R6.1 R27.2 R28.2 R29.2 R30.2 R31.1 R32.2 R48.2 R49.2 R50.2 R53.1 R71.2 R72.2 R73.2 R74.2 R75.1 R96.1 X5.2
-12V: C68.2 DC1.4(-VOUT) R26.1 R52.1 R70.1 R92.1
GND: B3.- C2.1 C3.1 C5.1 C7.1 C8.2 C9.2 C10.2 C12.1 C13.1 C15.1 C18.2 C19.2 C20.2 C21.1 C22.1 C24.1 C26.2 C27.2 C28.2 C30.1 C31.1 C33.1 C35.2 C36.2 C37.2 C38.2 C39.2 C40.1 C41.- C42.1 C43.- C44.1 C45.- C46.1 C47.- C48.1 C49.- C50.1 C51.2 C52.2 C53.- C54.2 C55.2 C56.2 C57.2 C58.- C59.- C60.1 C64.+ C66.2 C67.2 C68.1 C69.1 C70.1 C71.2 C72.1 C73.2 C74.2 C75.2 C76.- C77.2 C86.- C87.2 C88.- D3.A D4.A D7.A D8.A D11.A D12.A D15.A D16.A D19.A D20.A D23.A D24.A D27.A D28.A D31.A D32.A D33.A D45.A D52.A D54.A DC1.2(-VIN) DC1.5(COM) IC1.8(GND) IC2.8(GND) IC3.3(A:+IN) IC3.5(B:+IN) IC3.10(C:+IN) IC3.12(D:+IN) IC4.8(GND) IC5.8(GND) IC6.3(A:+IN) IC6.5(B:+IN) IC6.10(C:+IN) IC6.12(D:+IN) IC7.8(GND) IC8.8(GND) IC9.3(A:+IN) IC9.5(B:+IN) IC9.10(C:+IN) IC9.12(D:+IN) IC10.8(GND) IC11.8(GND) IC12.3(A:+IN) IC12.5(B:+IN) IC12.10(C:+IN) IC12.12(D:+IN) IC13.16(GND) IC14.16(GND) IC15.1(GND) IC15.2(GOE0) IC15.23(GND) IC16.1(OC) IC16.10(GND) IC17.10(GND) IC18.10(GND) IC19.14 IC20.1(OC) IC20.10(GND) IC21.10(GND) IC22.9(GND) IC23.2(!EA!) IC23.3(NMI) IC23.4(P0.3) IC23.5(P0.1) IC23.6(P0.0) IC23.7(P0.2) IC23.8(P0.6) IC23.9(P0.7) IC23.10(P0.5) IC23.11(P0.4) IC23.12(ANGND) IC23.14(VSS) IC23.24(HSI.0) IC23.25(HSI.1) IC23.26(HSI.2/HSO.4) IC23.27(HSI.3/HSI.5) IC23.36(VSS) IC23.68(VSS) IC25.5 IC25.6 IC25.7 IC26.3(GND) IC26.4(PFI) IC27.15(GND) JP1.1 LSP1.MP OK1.3(E) OK2.5(B:EMIT) OK2.7(A:EMIT) OK3.4(B:C) OK3.5(B:EMIT) OK3.7(A:EMIT) OK4.5(B:EMIT) OK4.7(A:EMIT) OK5.5(B:EMIT) OK5.7(A:EMIT) OK6.9(A:EMIT) OK6.11(B:EMIT) OK6.13(C:EMIT) OK6.15(D:EMIT) OK7.5(A:GND) OK9.5(A:GND) QF1.2 R7.1 R9.1 R23.2 R33.1 R35.1 R54.1 R56.1 R76.1 R78.1 R102.2 R103.2 R116.1 R126.2 SV1.2 SV2.2 SV5.1 SV6.2 SV7.2 U1.1(AGND) U1.5(DGND) U2.1(AGND) U2.5(DGND) U3.1(AGND) U3.5(DGND) U4.1(AGND) U4.5(DGND) U$1.2(A) X5.1 X14.5
GND1: B2.- C82.- C83.2 C84.- C85.2 D49.A D51.A IC29.GND OK2.2(A:C) OK2.4(B:C) OK3.2(A:C) X15.8
N$1: IC1.13(CE1) IC2.13(CE1) R5.2
N$2: D2.A D4.C IC1.15(OUT2) X1.2
N$3: D5.A D7.C IC2.1(OUT1) X1.3
N$4: D6.A D8.C IC2.15(OUT2) X1.4
N$5: IC1.5(OUTPUT-C.S.A) R10.2
N$6: D6.C IC2.14(RS2) R4.1
N$7: D1.A D3.C IC1.1(OUT1) X1.1
N$8: IC1.11(OSCILL.(R)) R7.2 R8.1
N$9: D2.C IC1.14(RS2) R2.1
N$10: D5.C IC2.2(RS1) R3.1
N$11: D1.C IC1.2(RS1) R1.1
N$12: C1.2 IC1.4(COMP.INPUT) R8.2
N$13: C1.1 C2.2 IC2.4(COMP.INPUT) IC2.10(OSCILL.(C))
N$14: IC2.11(OSCILL.(R)) R9.2
N$15: IC1.12(CE2) IC2.12(CE2) IC4.12(CE2) IC5.12(CE2) IC7.12(CE2) IC8.12(CE2) IC10.12(CE2) IC11.12(CE2) OK1.4(C) R6.2
N$16: C3.2 R10.1 R11.1
N$17: IC1.7(INPUT(ERR.AMPL.)) R11.2 R12.2
N$18: C4.1 R12.1
N$19: C4.2 IC1.9(OUTPUT(ERR.AMPL.))
N$20: IC2.5(OUTPUT-C.S.A) R13.2
N$21: C5.2 R13.1 R14.1
N$22: IC2.7(INPUT(ERR.AMPL.)) R14.2 R15.2
N$23: C6.1 R15.1
N$24: C6.2 IC2.9(OUTPUT(ERR.AMPL.))
N$25: IC1.6(INPUT) IC3.7(B:OUT) R16.2
N$26: IC3.6(B:-IN) R16.1 R17.2 R18.2
N$27: IC3.1(A:OUT) R17.1 U1.3(RFBA)
N$28: C7.2 R18.1 R20.1 R22.1 R24.2 R44.1 R46.1 R65.1 R67.1 R87.1 R89.1 U1.4(REFA) U1.18(REFB) U2.4(REFA) U2.18(REFB) U3.4(REFA) U3.18(REFB) U4.4(REFA) U4.18(REFB) U$1.3(C)
N$29: IC3.8(C:OUT) R19.1 U1.19(RFBB)
N$30: IC3.13(D:-IN) R19.2 R20.2 R21.1
N$31: IC2.6(INPUT) IC3.14(D:OUT) R21.2
N$32: IC3.2(A:-IN) U1.2(OUTA)
N$33: IC3.9(C:-IN) U1.20(OUTB)
N$34: C9.1 IC3.4(P:V+) R25.2
N$35: R22.2 R23.1 U$1.1(REF)
N$36: D10.A D12.C IC4.15(OUT2) X2.2
N$37: D13.A D15.C IC5.1(OUT1) X2.3
N$38: C8.1 IC3.11(P:V-) R26.2
N$39: D14.A D16.C IC5.15(OUT2) X2.4
N$40: D14.C IC5.14(RS2) R30.1
N$41: D13.C IC5.2(RS1) R29.1
N$42: D9.A D11.C IC4.1(OUT1) X2.1
N$43: D10.C IC4.14(RS2) R28.1
N$44: D9.C IC4.2(RS1) R27.1
N$45: IC4.13(CE1) IC5.13(CE1) R31.2
N$46: IC4.11(OSCILL.(R)) R33.2 R34.1
N$47: C11.2 IC4.4(COMP.INPUT) R34.2
N$48: C11.1 C12.2 IC5.4(COMP.INPUT) IC5.10(OSCILL.(C))
N$49: IC5.11(OSCILL.(R)) R35.2
N$50: OK1.1(A) R93.2
N$51: IC4.5(OUTPUT-C.S.A) R36.2
N$52: C13.2 R36.1 R37.1
N$53: IC4.7(INPUT(ERR.AMPL.)) R37.2 R38.2
N$54: C14.1 R38.1
N$55: C14.2 IC4.9(OUTPUT(ERR.AMPL.))
N$56: IC5.5(OUTPUT-C.S.A) R39.2
N$57: C15.2 R39.1 R40.1
N$58: IC5.7(INPUT(ERR.AMPL.)) R40.2 R41.2
N$59: C16.1 R41.1
N$60: C16.2 IC5.9(OUTPUT(ERR.AMPL.))
N$61: IC4.6(INPUT) IC6.7(B:OUT) R42.2
N$62: IC6.6(B:-IN) R42.1 R43.2 R44.2
N$63: IC6.1(A:OUT) R43.1 U2.3(RFBA)
N$64: R95.1 X1.9
N$65: IC6.8(C:OUT) R45.1 U2.19(RFBB)
N$66: IC6.13(D:-IN) R45.2 R46.2 R47.1
N$67: IC5.6(INPUT) IC6.14(D:OUT) R47.2
N$68: IC6.2(A:-IN) U2.2(OUTA)
N$69: IC6.9(C:-IN) U2.20(OUTB)
N$70: D18.A D20.C IC7.15(OUT2) X3.2
N$71: C19.1 IC6.4(P:V+) R51.2
N$72: C18.1 IC6.11(P:V-) R52.2
N$73: D21.A D23.C IC8.1(OUT1) X3.3
N$74: D22.A D24.C IC8.15(OUT2) X3.4
N$75: D22.C IC8.14(RS2) R50.1
N$76: D21.C IC8.2(RS1) R49.1
N$77: D17.A D19.C IC7.1(OUT1) X3.1
N$78: D18.C IC7.14(RS2) R48.1
N$79: D17.C IC7.2(RS1) R32.1
N$80: IC7.13(CE1) IC8.13(CE1) R53.2
N$81: IC7.11(OSCILL.(R)) R54.2 R55.1
N$82: C17.2 IC7.4(COMP.INPUT) R55.2
N$83: C17.1 C21.2 IC8.4(COMP.INPUT) IC8.10(OSCILL.(C))
N$84: IC8.11(OSCILL.(R)) R56.2
N$85: IC7.5(OUTPUT-C.S.A) R57.2
N$86: C22.2 R57.1 R58.1
N$87: IC7.7(INPUT(ERR.AMPL.)) R58.2 R59.2
N$88: C23.1 R59.1
N$89: C23.2 IC7.9(OUTPUT(ERR.AMPL.))
N$90: IC8.5(OUTPUT-C.S.A) R60.2
N$91: C24.2 R60.1 R61.1
N$92: IC8.7(INPUT(ERR.AMPL.)) R61.2 R62.2
N$93: C25.1 R62.1
N$94: C25.2 IC8.9(OUTPUT(ERR.AMPL.))
N$95: IC7.6(INPUT) IC9.7(B:OUT) R63.2
N$96: IC9.6(B:-IN) R63.1 R64.2 R65.2
N$97: IC9.1(A:OUT) R64.1 U3.3(RFBA)
N$98: IC9.8(C:OUT) R66.1 U3.19(RFBB)
N$99: IC9.13(D:-IN) R66.2 R67.2 R68.1
N$100: IC8.6(INPUT) IC9.14(D:OUT) R68.2
N$101: IC9.2(A:-IN) U3.2(OUTA)
N$102: IC9.9(C:-IN) U3.20(OUTB)
N$103: C27.1 IC9.4(P:V+) R69.2
N$104: C26.1 IC9.11(P:V-) R70.2
N$105: D26.A D28.C IC10.15(OUT2) X4.2
N$106: D29.A D31.C IC11.1(OUT1) X4.3
N$107: D30.A D32.C IC11.15(OUT2) X4.4
N$108: D30.C IC11.14(RS2) R74.1
N$109: D29.C IC11.2(RS1) R73.1
N$110: D25.A D27.C IC10.1(OUT1) X4.1
N$111: D26.C IC10.14(RS2) R72.1
N$112: D25.C IC10.2(RS1) R71.1
N$113: IC10.13(CE1) IC11.13(CE1) R75.2
N$114: IC10.11(OSCILL.(R)) R76.2 R77.1
N$115: C29.2 IC10.4(COMP.INPUT) R77.2
N$116: C29.1 C30.2 IC11.4(COMP.INPUT) IC11.10(OSCILL.(C))
N$117: IC11.11(OSCILL.(R)) R78.2
N$118: IC10.5(OUTPUT-C.S.A) R79.2
N$119: C31.2 R79.1 R80.1
N$120: IC10.7(INPUT(ERR.AMPL.)) R80.2 R81.2
N$121: C32.1 R81.1
N$122: C32.2 IC10.9(OUTPUT(ERR.AMPL.))
N$123: IC11.5(OUTPUT-C.S.A) R82.2
N$124: C33.2 R82.1 R83.1
N$125: IC11.7(INPUT(ERR.AMPL.)) R83.2 R84.2
N$126: C34.1 R84.1
N$127: C34.2 IC11.9(OUTPUT(ERR.AMPL.))
N$128: IC10.6(INPUT) IC12.7(B:OUT) R85.2
N$129: IC12.6(B:-IN) R85.1 R86.2 R87.2
N$130: IC12.1(A:OUT) R86.1 U4.3(RFBA)
N$131: IC12.8(C:OUT) R88.1 U4.19(RFBB)
N$132: IC12.13(D:-IN) R88.2 R89.2 R90.1
N$133: IC11.6(INPUT) IC12.14(D:OUT) R90.2
N$134: IC12.2(A:-IN) U4.2(OUTA)
N$135: IC12.9(C:-IN) U4.20(OUTB)
N$136: C36.1 IC12.4(P:V+) R91.2
N$137: C35.1 IC12.11(P:V-) R92.2
N$138: R94.1 X1.7
N$139: R97.1 X2.9
N$140: IC13.13(O0) IC16.2(1D) IC23.52(P4.0) RN1.2 U1.14(DB0) U2.14(DB0)
N$141: R98.1 X3.7
N$142: R99.1 X3.9
N$143: JP2.1 R100.1 X4.7
N$144: R101.1 X4.9
N$145: OK4.1(A:A) R99.2
N$146: OK4.3(B:A) R98.2
N$147: OK2.1(A:A) R95.2
N$148: OK2.3(B:A) R94.2
N$149: OK3.1(A:A) R97.2
N$150: OK3.3(B:A) R96.2
N$151: OK5.1(A:A) R101.2
N$152: OK5.3(B:A) R100.2
N$153: B1.AC2 F3.2A
N$154: B1.AC1 X15.2
N$155: IC13.14(O1) IC16.3(2D) IC23.51(P4.1) RN1.3 U1.13(DB1) U2.13(DB1)
N$156: IC13.15(O2) IC16.4(3D) IC23.50(P4.2) RN1.4 U1.12(DB2) U2.12(DB2)
N$157: IC13.17(O3) IC16.5(4D) IC23.49(P4.3) RN1.5 U1.11(DB3) U2.11(DB3)
N$158: IC13.18(O4) IC16.6(5D) IC23.48(P4.4) RN1.6 U1.10(DB4) U2.10(DB4)
N$159: IC13.19(O5) IC16.7(6D) IC23.47(P4.5) RN1.7 U1.9(DB5) U2.9(DB5)
N$160: IC13.20(O6) IC16.8(7D) IC23.46(P4.6) RN1.8 U1.8(DB6) U2.8(DB6)
N$161: IC13.21(O7) IC16.9(8D) IC23.45(P4.7) RN1.9 U1.7(DB7) U2.7(DB7)
N$162: IC14.13(O0) IC17.18(Y1) IC18.18(Y1) IC19.11 IC20.2(1D) IC21.3(D1) IC23.60(P3.0) RN4.2 U3.14(DB0) U4.14(DB0)
N$163: IC14.14(O1) IC17.17(Y2) IC18.17(Y2) IC19.12 IC20.3(2D) IC21.4(D2) IC23.59(P3.1) RN4.3 U3.13(DB1) U4.13(DB1)
N$164: IC14.15(O2) IC17.16(Y3) IC18.16(Y3) IC19.13 IC20.4(3D) IC21.7(D3) IC23.58(P3.2) RN4.4 U3.12(DB2) U4.12(DB2)
N$165: IC14.17(O3) IC17.15(Y4) IC18.15(Y4) IC19.15 IC20.5(4D) IC21.8(D4) IC23.57(P3.3) RN4.5 U3.11(DB3) U4.11(DB3)
N$166: IC14.18(O4) IC17.14(Y5) IC18.14(Y5) IC19.16 IC20.6(5D) IC21.13(D5) IC23.56(P3.4) RN4.6 U3.10(DB4) U4.10(DB4)
N$167: IC14.19(O5) IC17.13(Y6) IC18.13(Y6) IC19.17 IC20.7(6D) IC21.14(D6) IC23.55(P3.5) RN4.7 U3.9(DB5) U4.9(DB5)
N$168: IC14.20(O6) IC17.12(Y7) IC18.12(Y7) IC19.18 IC20.8(7D) IC21.17(D7) IC23.54(P3.6) RN4.8 U3.8(DB6) U4.8(DB6)
N$169: IC14.21(O7) IC17.11(Y8) IC18.11(Y8) IC19.19 IC20.9(8D) IC21.18(D8) IC23.53(P3.7) RN4.9 U3.7(DB7) U4.7(DB7)
N$170: IC15.5(IO26) IC21.11(CLK)
N$171: IC13.12(A0) IC14.12(A0) IC19.9 IC20.18(2Q) U1.6(DA/DB) U2.6(DA/DB) U3.6(DA/DB) U4.6(DA/DB)
N$172: IC15.10(IO31) U1.15(CS) U3.15(CS)
N$173: IC15.9(IO30) U2.15(CS) U4.15(CS)
N$174: IC13.31(WE/) IC23.41(!BHE!/!WRH!) U1.16(WR) U2.16(WR)
N$175: IC14.31(WE/) IC15.28(IO11) IC19.27 IC23.40(!WR!/!WRL!) U3.16(WR) U4.16(WR)
N$176: IC13.4(A12) IC14.4(A12) IC15.20(IO5) IC16.14(6Q)
N$177: IC13.5(A7) IC14.5(A7) IC15.27(IO10) IC16.19(1Q) IC19.25
N$178: IC13.2(A16) IC14.2(A16) IC23.34(HSO.2) R102.1
N$179: IC13.3(A15) IC14.3(A15) R103.1 SV3.2
N$180: IC13.29(A14) IC14.29(A14) IC15.18(IO3) IC16.12(8Q)
N$181: IC13.28(A13) IC14.28(A13) IC15.19(IO4) IC16.13(7Q)
N$182: IC13.6(A6) IC14.6(A6) IC19.3 IC20.12(8Q)
N$183: IC13.25(A11) IC14.25(A11) IC15.21(IO6) IC16.15(5Q)
N$184: IC13.23(A10) IC14.23(A10) IC15.22(IO7) IC16.16(4Q)
N$185: IC13.26(A9) IC14.26(A9) IC15.25(IO8) IC16.17(3Q) IC19.21
N$186: IC13.27(A8) IC14.27(A8) IC15.26(IO9) IC16.18(2Q) IC19.24
N$187: IC13.7(A5) IC14.7(A5) IC19.4 IC20.13(7Q)
N$188: IC13.8(A4) IC14.8(A4) IC19.5 IC20.14(6Q)
N$189: IC13.9(A3) IC14.9(A3) IC19.6 IC20.15(5Q)
N$190: IC13.10(A2) IC14.10(A2) IC19.7 IC20.16(4Q)
N$191: IC13.11(A1) IC14.11(A1) IC19.8 IC20.17(3Q)
N$192: IC13.24(!OE) IC14.24(!OE) IC17.19(G2) IC18.19(G2) IC19.22
N$196: B2.AC1 X15.6
N$197: IC17.9(A8) OK5.8(A:COL) RN2.9
N$198: IC17.8(A7) OK5.6(B:COL) RN2.8
N$199: IC17.7(A6) OK4.8(A:COL) RN2.7
N$200: IC17.6(A5) OK4.6(B:COL) RN2.6
N$201: IC17.5(A4) OK3.8(A:COL) RN2.5
N$202: IC15.39(IO18) IC17.4(A3) OK3.6(B:COL) RN2.4
N$203: IC17.3(A2) OK2.8(A:COL) RN2.3
N$204: IC17.2(A1) OK2.6(B:COL) RN2.2
N$205: IC19.10 IC20.19(1Q)
N$206: C72.2 IC16.11(C) IC20.11(C) IC23.62(ALE/!ADV!)
N$207: IC15.43(IO22) IC19.23
N$208: IC15.8(IO29) IC19.20
N$209: OK6.1(A:A) R104.1
N$210: IC15.16(IO1) IC19.1 IC23.43(READY)
N$211: IC15.41(IO20) IC19.2
N$212: IC13.22(!CE) IC14.22(!CE) IC15.17(IO2)
N$213: IC18.9(A8) IC23.33(P2.6/T2U-D) OK7.6(B:VO2) RN3.9
N$214: IC18.8(A7) IC23.42(P2.4/T2RST) OK7.7(A:VO1) RN3.8
N$215: IC18.7(A6) IC23.44(P2.3/T2CLK) OK9.6(B:VO2) RN3.7
N$216: IC18.6(A5) JP1.2 OK9.7(A:VO1) RN3.6
N$217: IC18.5(A4) OK6.10(A:COL) RN3.5
N$218: IC18.4(A3) OK6.12(B:COL) RN3.4
N$219: IC18.3(A2) OK6.14(C:COL) RN3.3
N$220: IC15.32(IO15) IC18.2(A1) OK6.16(D:COL) RN3.2
N$221: IC15.11(Y0) IC15.35(Y1/!RESET) IC21.1(CLR) IC23.16(!RESET!) U$2.A
N$222: IC15.6(IO27) IC18.1(G1)
N$223: IC15.7(IO28) IC17.1(G1)
N$224: IC15.33(Y2/SCLK) RN5.3 SV1.1
N$225: IC15.14(IN0/SDI) RN5.5 SV1.6
N$226: IC15.13(!ISPEN) RN5.7 SV1.5
N$227: OK6.3(B:A) R105.1
N$228: IC15.36(IN2/MODE) RN5.6 SV1.3
N$229: IC15.24(IN1/SDO) RN5.4 SV1.7
N$230: OK6.5(C:A) R106.1
N$231: OK6.7(D:A) R107.1
N$232: D35.A K3.16 OK4.2(A:C) OK4.4(B:C) OK5.2(A:C) OK5.4(B:C) OK6.2(A:C) OK6.4(B:C) OK6.6(C:C) OK6.8(D:C) OK7.2(A:C1) OK7.3(B:C2) OK9.2(A:C1) OK9.3(B:C2) R113.1 X6.9 X7.1 X12.6 X12.7 X12.8 X12.9
N$233: OK9.4(B:A2) R108.1
N$234: OK9.1(A:A1) R109.1
N$235: OK7.4(B:A2) R110.1
N$236: OK7.1(A:A1) R111.1
N$237: R107.2 X6.1
N$238: OK8.6(B:COL) OK8.8(A:COL) X6.6 X6.7 X6.8 X7.2 X10.5 X12.1 X12.5
N$239: R106.2 X6.2
N$240: R105.2 X6.3
N$241: R104.2 X6.4
N$242: R109.2 X9.8
N$243: R108.2 X9.7
N$244: R110.2 X9.6
N$245: K1.S2(3:S) X8.2 X9.4 X9.5 X9.12 X10.3
N$246: R111.2 R113.2 X10.4
N$247: X9.9 X9.10
N$248: D34.A IC22.11(O8) K1.1
N$249: D34.C K1.2 K1.P1(2:P) K3.S1(2:S)
N$250: K1.P2(3:P) X10.1
N$251: C58.+ D38.C IC22.10(CD+) K1.S1(2:S) K2.S1(2:S) K3.P1(2:P) K5.1 R93.1 R114.1 R115.1 SV2.1
N$252: D35.C K3.1 X6.5
N$253: IC22.18(O1) OK1.2(K)
N$254: K2.P1(2:P) K2.S2(3:S)
N$255: K2.P2(3:P) K4.S1(2:S)
N$256: D36.A D37.A K2.2 K4.2 R112.2 X8.1 X10.6 X10.7 X10.8 X10.9 X11.2
N$257: K4.S2(3:S) K5.S1(2:S) X9.1
N$258: D36.C D39.A K4.1 K4.P2(3:P) X11.1
N$259: D37.C K2.1 X10.2
N$260: K5.P1(2:P) X9.2
N$261: D38.A IC22.17(O2) K5.2
N$262: D39.K(C) R112.1
N$263: OK8.1(A:A) R114.2
N$264: D42.K(C) IC22.16(O3)
N$265: D41.K(C) IC22.15(O4)
N$266: IC22.13(O6) OK8.2(A:C)
N$267: IC22.12(O7) OK8.4(B:C)
N$268: D43.C D44.C K4.P1(2:P) K6.3(A) K7.3(A) K8.3(A) K9.A1 K10.A1 R116.2
N$269: D40.K(C) IC22.14(O5)
N$270: D41.A D43.A K7.4(K) K9.A2
N$271: D42.A D44.A K8.4(K) K10.A2
N$272: F2.1A F2.1B K6.2(DS2) K7.2(DS2) K9.11(2:P) K9.21(3:P) K9.22(3:O)
N$273: D40.A K6.4(K)
N$274: K7.1(DS1) K9.14(2:S) K9.24(3:S) R119.1 X13.6
N$275: K8.2(DS2) K10.11(2:P) K10.21(3:P) R118.1 X13.7
N$276: F1.1A F1.1B K8.1(DS1) K10.14(2:S) K10.24(3:S)
N$277: OK8.3(B:A) R115.2
N$278: F1.2A F1.2B F2.2A F2.2B X13.8
N$279: OK8.5(B:EMIT) X12.3
N$280: OK8.7(A:EMIT) X12.2
N$281: R117.1 R118.2 R119.2 X13.2 X13.3 X13.4 X13.5
N$282: K6.1(DS1) R117.2 X13.1
N$283: IC21.2(Q1) IC22.1(I1)
N$284: IC21.5(Q2) IC22.2(I2)
N$285: IC21.6(Q3) IC22.3(I3)
N$286: IC21.9(Q4) IC22.4(I4)
N$287: IC21.12(Q5) IC22.5(I5)
N$288: IC21.15(Q6) IC22.6(I6)
N$289: IC21.16(Q7) IC22.7(I7)
N$290: IC21.19(Q8) IC22.8(I8)
N$291: IC23.35(HSO.3) SV3.1
N$292: IC15.15(IO0) IC23.64(BUSWIDTH)
N$293: IC23.39(P2.5/PWM0) IC24.2
N$294: IC24.4 R120.2
N$295: IC24.1 R121.2
N$296: IC24.7 SV4.2
N$297: IC23.29(HSO.1) IC24.3
N$298: IC24.8 SV4.4
N$299: C61.1 IC24.5 SV4.3 SV5.3
N$300: IC24.6 SV4.1
N$301: C61.2 SV5.4
N$302: IC23.31(P1.6/!HLDA!) IC25.2 SV6.9
N$303: IC25.3 IC25.4 R122.1
N$304: IC23.30(P1.5/!BREQ!) R122.2 SV6.8
N$305: IC23.32(P1.7/!HOLD!) IC25.1 SV6.10
N$306: IC26.1(MR) IC26.8(WDO)
N$307: IC26.7(RESET) U$2.C
N$308: IC23.28(HSO.0) IC26.6(WDI)
N$309: IC27.13(R1IN) X14.4
N$310: IC27.14(T1OUT) X14.3
N$311: IC23.17(P2.1/RXD) IC27.12(R1OUT)
N$312: IC23.18(P2.0/TXD) IC27.11(T1IN)
N$313: C62.- IC27.3(C1-)
N$314: C62.+ IC27.1(C1+)
N$315: C63.+ IC27.4(C2+)
N$316: C63.- IC27.5(C2-)
N$317: C64.- IC27.6(V-)
N$318: IC15.42(IO21) IC23.15(P2.2/!PROG!)
N$319: C65.+ IC27.2(V+)
N$320: IC23.19(P1.0) SV6.3
N$321: IC23.20(P1.1) SV6.4
N$322: IC23.21(P1.2) SV6.5
N$323: IC23.22(P1.3/PWM1) SV6.6
N$324: IC23.23(P1.4/PWM2) SV6.7
N$325: C70.2 IC23.67(X1) QF1.3
N$326: C69.2 IC23.66(X2) QF1.1
N$327: F3.1A X15.1
N$328: B2.AC2 F4.2A
N$329: F5.1A X15.9
N$330: B1.+ C78.+ C79.1 D46.C D50.C IC28.IN
N$331: B1.- C78.- C79.2 C80.- C81.2 D47.A D50.A IC28.GND X15.4
N$332: D47.K(C) R123.2
N$333: C80.+ C81.1 D46.A IC28.OUT R123.1 X15.3
N$334: F4.1A X15.5
N$335: B2.+ C82.+ C83.1 D48.C D51.C IC29.IN
N$336: B3.AC1 F5.2A
N$337: B3.AC2 X15.10
N$338: B3.+ C86.+ C87.1 D52.C D53.C IC30.3(IN) R24.1 R127.1 SV7.1
N$339: D54.K(C) R127.2
N$340: D49.K(C) R124.2
N$342: IC30.1(ADJ) R125.2 R126.1
Unconnected: F3.1B F3.2B F4.1B F4.2B F5.1B F5.2B IC1.10(OSCILL.(C)) IC4.10(OSCILL.(C)) IC7.10(OSCILL.(C)) IC10.10(OSCILL.(C)) IC13.1(NC) IC14.1(NC) IC15.3(IO24) IC15.4(IO25) IC15.29(IO12) IC15.30(IO13) IC15.31(IO14) IC15.37(IO16) IC15.38(IO17) IC15.40(IO19) IC15.44(IO23) IC23.13(VREF) IC23.38(P2.7/T2CAP) IC23.61(!RD!) IC23.63(INST) IC23.65(CLKOUT) IC26.5(PFO) IC27.7(T2OUT) IC27.8(R2IN) IC27.9(R2OUT) IC27.10(T2IN) K1.O1(2:O) K1.O2(3:O) K2.O1(2:O) K2.O2(3:O) K3.O1(2:O) K3.O2(3:O) K3.P2(3:P) K3.S2(3:S) K4.O1(2:O) K4.O2(3:O) K5.O1(2:O) K5.O2(3:O) K5.P2(3:P) K5.S2(3:S) K9.12(2:O) K10.12(2:O) K10.22(3:O) RN5.2 SV1.4 SV2.3 SV7.3 X1.6 X1.8 X2.6 X2.7 X2.8 X3.6 X3.8 X4.6 X4.8 X9.3 X9.11 X9.13 X9.14 X9.15 X9.G1 X9.G2 X12.4 X14.1 X14.2 X14.6 X14.7 X14.8 X14.9

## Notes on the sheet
- Isel IMC4 Schaltplan
- Y
- A
- X
- Z
- Gabs'e 2015
- !!! ACHTUNG Es wird keine Haftung für die
   Richtigkeit von Schaltplan und Layout übernommen !!!

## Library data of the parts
B1 B2 = rectifier:RECTIFIER-: Rectifier
B3 = rectifier:2KBB-R: RECTIFIER grid 3 x 5 mm
C1-C40 C42 C44 C46 C48 C50-C52 C54-C57 C60 C61 C66-C75 C77 C79 C81 C83 C85 C87 = rcl:C-EU: CAPACITOR, European symbol
C41 C43 C45 C47 C49 C53 C58 C59 C62-C65 C76 C78 C80 C82 C84 C86 C88 = rcl:CPOL-EU: POLARIZED CAPACITOR, European symbol
D1-D32 = diode:MUR150RL: DIODE
D33 = diode:1N5060GP: DIODE
D34-D38 D43 D44 = Gabse:1N4004: DIODE
D39-D42 D47 D49 D54 = led:U57X32: LED
D45 D50 D51 = diode:P6KEXXA: DIODE
D46 D48 D53 = diode:1N4004: DIODE
D52 = Gabse:BZW06-28: DIODE
DC1 = dc-dc-converter:NMA: DC-DC CONVERTER; MF: C & D TECHNOLOGIES, INC; MPN: NMA0515SC; OC_FARNELL: 1021434; OC_NEWARK: 61K3064
F1-F5 = fuse:SHK20L: FUSE HOLDER 5 x 20 mm, SH contact, SHH1 Schukat, E1073 Buerklin; OC_FARNELL: unknown; OC_NEWARK: unknown
IC1 IC2 IC4 IC5 IC7 IC8 IC10 IC11 = Gabse:L292: SWITCH-MODE DRIVER FOR DC MOTORS
IC3 IC6 IC9 IC12 = Gabse:TLE2064: OP AMP
IC13 IC14 = am29-memory:AM29F010*: 1-Megabit FLASH MEMORY (128 K x 8 bit) 5 V-only
IC15 = Gabse:LSI2032: LATTICE PROGRAMMABLE DEVICE
IC16 IC20 = 74xx-eu:74*573: 8-bit D latch BUS DRIVER
IC17 IC18 = 74xx-eu:74*540: Octal BUFFER and LINE DRIVER, 3-state
IC19 = ic-package:DIL28: Dual In Line
IC21 = 74xx-eu:74*273: Octal D type FLIP FLOP, clear
IC22 = uln-udn:ULN2803A: DRIVER ARRAY
IC23 = Gabse:N80C196KC: MICROCOMPUTER/PERIPHERAL DEVICE
IC24 IC25 = ic-package:DIL8: Dual In Line / Socket
IC26 = maxim:MAX705CPA: WATCHDOG; MPN: MAX705CPA; OC_FARNELL: 9726004; OC_NEWARK: 34C4002
IC27 = maxim:MAX232: RS232 TRANSCEIVER; MF: MAXIM; MPN: MAX232ACPE+; OC_FARNELL: 9723773; OC_NEWARK: 68K4544
IC28 IC29 = v-reg:78XXS: VOLTAGE REGULATOR
IC30 = v-reg:LM317TS: VOLTAGE REGULATOR
JP1 JP2 = pinhead:PINHD-1X2: PIN HEADER
K1 K2 K4 K5 = relay:4052: RELAY 2 x switch, Finder; OC_FARNELL: unknown; OC_NEWARK: unknown
K3 = relay:351: RELAY 2 x switch, Omron; OC_FARNELL: unknown; OC_NEWARK: unknown
K6-K8 = relay:AQ?: SOLID STATE RELAY NAiS Source: http://www.mew-europe.com/.. en_ds_61601_0000.pdf; MPN: AQ2A2-ZP3/28VDC; OC_FARNELL: 1163552; OC_NEWARK: 13P1232
K9 K10 = relay:RT424A*: Power PCB Relay polarized bistable version SCHRACK 2 pole 8 A Source: http://www.schrack.com/.. 5843.pdf; MPN: RT424A12; OC_FARNELL: unknown; OC_NEWARK: 48M7977
LSP1 = solpad:LSP10: SOLDER PAD
OK1 = Gabse:TLP523: MOTOROLA OPTO COUPLER; MF: AGILENT TECHNOLOGIES; MPN: 4N45; OC_FARNELL: unknown; OC_NEWARK: 09F6959
OK2-OK5 OK8 = optocoupler:ILD621: SIEMENS OPTO COUPLER; MF: VISHAY/TELEFUNKEN; MPN: ILD621; OC_FARNELL: 1020151; OC_NEWARK: 58K1678
OK6 = Gabse:TLP621-4: SIEMENS OPTO COUPLER
OK7 OK9 = optocoupler:HCPL2530: HEWLETT PACKARD OPTO COUPLER; MF: AGILENT TECHNOLOGIES; MPN: HCPL-2530-000E; OC_FARNELL: 9994793; OC_NEWARK: 31K6974
QF1 = crystal:8M10AHC49T: Monolithic Crystal Filters Source: www.vanlong.com; OC_FARNELL: unknown; OC_NEWARK: unknown
R1-R116 R120-R127 = rcl:R-EU_: RESISTOR, European symbol
R117-R119 = varistor:S20K250: VARISTOR
RN1-RN4 = resistor-net:RN08: RESISTOR NETWORK; OC_FARNELL: unknown; OC_NEWARK: unknown
RN5 = resistor-net:RN06: RESISTOR NETWORK; OC_FARNELL: unknown; OC_NEWARK: unknown
SV1 = con-lstb:MA04-2: PIN HEADER; OC_FARNELL: unknown; OC_NEWARK: unknown
SV2 SV3 SV7 = con-lstb:MA03-1: PIN HEADER; OC_FARNELL: unknown; OC_NEWARK: unknown
SV4 SV5 = con-lstb:MA04-1: PIN HEADER; OC_FARNELL: unknown; OC_NEWARK: unknown
SV6 = con-lstb:MA05-2: PIN HEADER; OC_FARNELL: unknown; OC_NEWARK: unknown
U1-U4 = Gabse:TLC7528: DIGITAL-TO-ANALOG CONVERTER
U$1 = GuShH:TL431
U$2 = Gabse:SB030: Miniature Schottky Barrier Rectifier
X1-X4 X6 X10 X12 X14 = con-subd:F09: SUB-D; OC_FARNELL: unknown; OC_NEWARK: unknown
X5 X7 X8 X11 = con-wago-508:W237-02P: WAGO SREW CLAMP; OC_FARNELL: unknown; OC_NEWARK: unknown
X9 = con-subd:F15VP: SUB-D; OC_FARNELL: unknown; OC_NEWARK: unknown
X13 = con-wago-508:W237-08P: WAGO SREW CLAMP; OC_FARNELL: unknown; OC_NEWARK: unknown
X15 = con-wago-508:W237-10P: WAGO SREW CLAMP; OC_FARNELL: unknown; OC_NEWARK: unknown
